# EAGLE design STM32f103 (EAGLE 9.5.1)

## Sheet 1 of 9: STM32F103C8TU
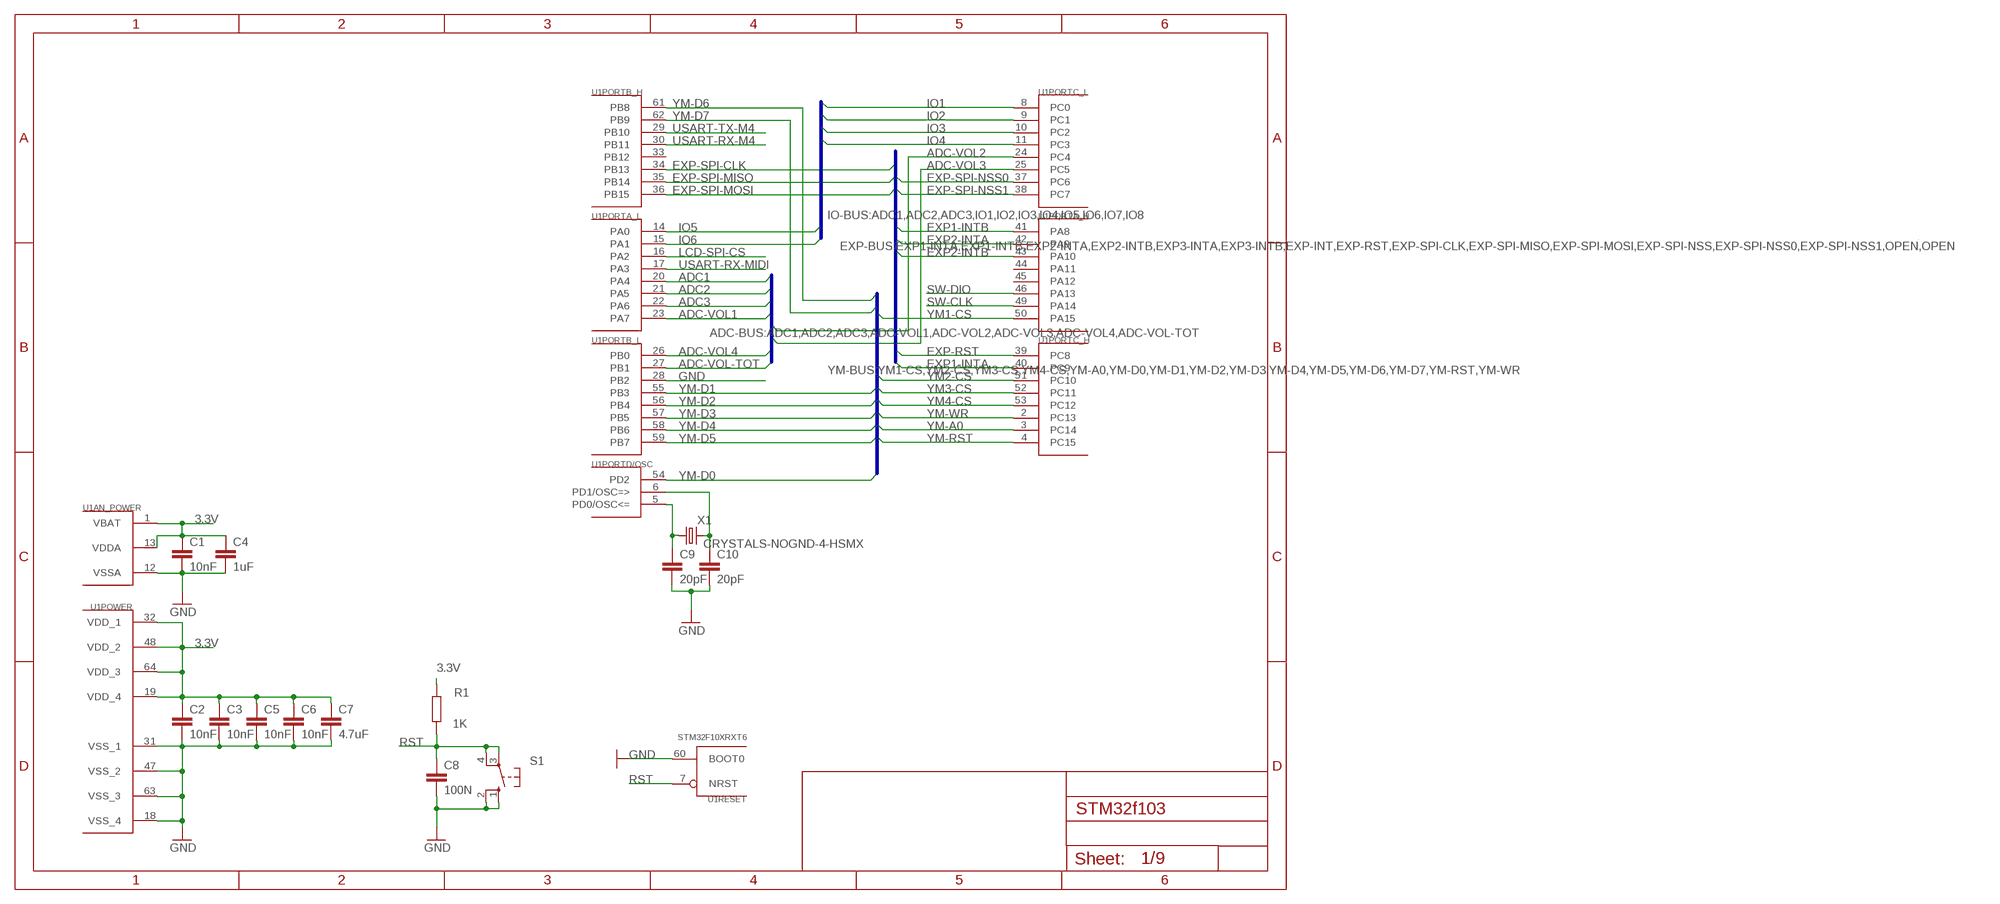
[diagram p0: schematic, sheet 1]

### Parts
C1  10nF  C-EUC0603  [C0603]
C2  10nF  C-EUC0603  [C0603]
C3  10nF  C-EUC0603  [C0603]
C4  1uF  C-EUC0603  [C0603]
C5  10nF  C-EUC0603  [C0603]
C6  10nF  C-EUC0603  [C0603]
C7  4.7uF  C-EUC0603  [C0603]
C8  100N  [0603-SMD]
C9  20pF  C-EUC0603  [C0603]
C10  20pF  C-EUC0603  [C0603]
R1  1K  [0805-SMD]
S1  10-XX  [B3F-10XX]
U1  STM32F10XRXT6  [TQFP64]
X1  CRYSTALS-NOGND-4-HSMX  [HC49-4-HSMX]

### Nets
3.3V: C1.1 C2.1 C3.1 C4.1 C5.1 C6.1 C7.1 R1.2 U1.1(AN_POWER:VBAT) U1.13(AN_POWER:VDDA) U1.19(POWER:VDD_4) U1.32(POWER:VDD_1) U1.48(POWER:VDD_2) U1.64(POWER:VDD_3) ; also sheet 6,9
ADC1: U1.20(PORTA_L:PA4) ; also sheet 9
ADC2: U1.21(PORTA_L:PA5) ; also sheet 9
ADC3: U1.22(PORTA_L:PA6) ; also sheet 9
ADC-VOL1: U1.23(PORTA_L:PA7) ; also sheet 9
ADC-VOL2: U1.24(PORTC_L:PC4) ; also sheet 9
ADC-VOL3: U1.25(PORTC_L:PC5) ; also sheet 9
ADC-VOL4: U1.26(PORTB_L:PB0) ; also sheet 9
ADC-VOL-TOT: U1.27(PORTB_L:PB1) ; also sheet 9
EXP1-INTA: U1.40(PORTC_H:PC9) ; also sheet 9
EXP1-INTB: U1.41(PORTA_H:PA8) ; also sheet 9
EXP2-INTA: U1.42(PORTA_H:PA9) ; also sheet 9
EXP2-INTB: U1.43(PORTA_H:PA10) ; also sheet 9
EXP-RST: U1.39(PORTC_H:PC8) ; also sheet 9
EXP-SPI-CLK: U1.34(PORTB_H:PB13) ; also sheet 9
EXP-SPI-MISO: U1.35(PORTB_H:PB14) ; also sheet 9
EXP-SPI-MOSI: U1.36(PORTB_H:PB15) ; also sheet 9
EXP-SPI-NSS0: U1.37(PORTC_L:PC6) ; also sheet 9
EXP-SPI-NSS1: U1.38(PORTC_L:PC7) ; also sheet 9
GND: C1.2 C2.2 C3.2 C4.2 C5.2 C6.2 C7.2 C8.2 C9.2 C10.2 S1.1(S) S1.2(S1) U1.12(AN_POWER:VSSA) U1.18(POWER:VSS_4) U1.28(PORTB_L:PB2) U1.31(POWER:VSS_1) U1.47(POWER:VSS_2) U1.60(RESET:BOOT0) U1.63(POWER:VSS_3) ; also sheet 2,3,4,5,6,7,8,9
IO1: U1.8(PORTC_L:PC0) ; also sheet 9
IO2: U1.9(PORTC_L:PC1) ; also sheet 9
IO3: U1.10(PORTC_L:PC2) ; also sheet 9
IO4: U1.11(PORTC_L:PC3) ; also sheet 9
IO5: U1.14(PORTA_L:PA0) ; also sheet 9
IO6: U1.15(PORTA_L:PA1) ; also sheet 9
LCD-SPI-CS: U1.16(PORTA_L:PA2) ; also sheet 9
N$1: C9.1 U1.5(PORTD/OSC:PD0/OSC<=) X1.1
N$2: C10.1 U1.6(PORTD/OSC:PD1/OSC=>) X1.2
RST: C8.1 R1.1 S1.3(P) S1.4(P1) U1.7(RESET:NRST)
SW-CLK: U1.49(PORTA_H:PA14) ; also sheet 9
SW-DIO: U1.46(PORTA_H:PA13) ; also sheet 9
USART-RX-M4: U1.30(PORTB_H:PB11) ; also sheet 9
USART-RX-MIDI: U1.17(PORTA_L:PA3) ; also sheet 7
USART-TX-M4: U1.29(PORTB_H:PB10) ; also sheet 9
YM1-CS: U1.50(PORTA_H:PA15) ; also sheet 2
YM2-CS: U1.51(PORTC_H:PC10) ; also sheet 3
YM3-CS: U1.52(PORTC_H:PC11) ; also sheet 4
YM4-CS: U1.53(PORTC_H:PC12) ; also sheet 5
YM-A0: U1.3(PORTC_H:PC14) ; also sheet 2,3,4,5
YM-D0: U1.54(PORTD/OSC:PD2) ; also sheet 2,3,4,5
YM-D1: U1.55(PORTB_L:PB3) ; also sheet 2,3,4,5
YM-D2: U1.56(PORTB_L:PB4) ; also sheet 2,3,4,5
YM-D3: U1.57(PORTB_L:PB5) ; also sheet 2,3,4,5
YM-D4: U1.58(PORTB_L:PB6) ; also sheet 2,3,4,5
YM-D5: U1.59(PORTB_L:PB7) ; also sheet 2,3,4,5
YM-D6: U1.61(PORTB_H:PB8) ; also sheet 2,3,4,5
YM-D7: U1.62(PORTB_H:PB9) ; also sheet 2,3,4,5
YM-RST: U1.4(PORTC_H:PC15) ; also sheet 2,3,4,5
YM-WR: U1.2(PORTC_H:PC13) ; also sheet 2,3,4,5
Unconnected: U1.33(PORTB_H:PB12) U1.44(PORTA_H:PA11) U1.45(PORTA_H:PA12)

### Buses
YM-BUS:YM1-CS,YM2-CS,YM3-CS,YM4-CS,YM-A0,YM-D0,YM-D1,YM-D2,YM-D3,YM-D4,YM-D5,YM-D6,YM-D7,YM-RST,YM-WR
EXP-BUS:EXP1-INTA,EXP1-INTB,EXP2-INTA,EXP2-INTB,EXP3-INTA,EXP3-INTB,EXP-INT,EXP-RST,EXP-SPI-CLK,EXP-SPI-MISO,EXP-SPI-MOSI,EXP-SPI-NSS,EXP-SPI-NSS0,EXP-SPI-NSS1,OPEN!,OPEN
IO-BUS:ADC1,ADC2,ADC3,IO1,IO2,IO3,IO4,IO5,IO6,IO7,IO8
ADC-BUS:ADC1,ADC2,ADC3,ADC-VOL1,ADC-VOL2,ADC-VOL3,ADC-VOL4,ADC-VOL-TOT

## Sheet 2 of 9: YM3812-0
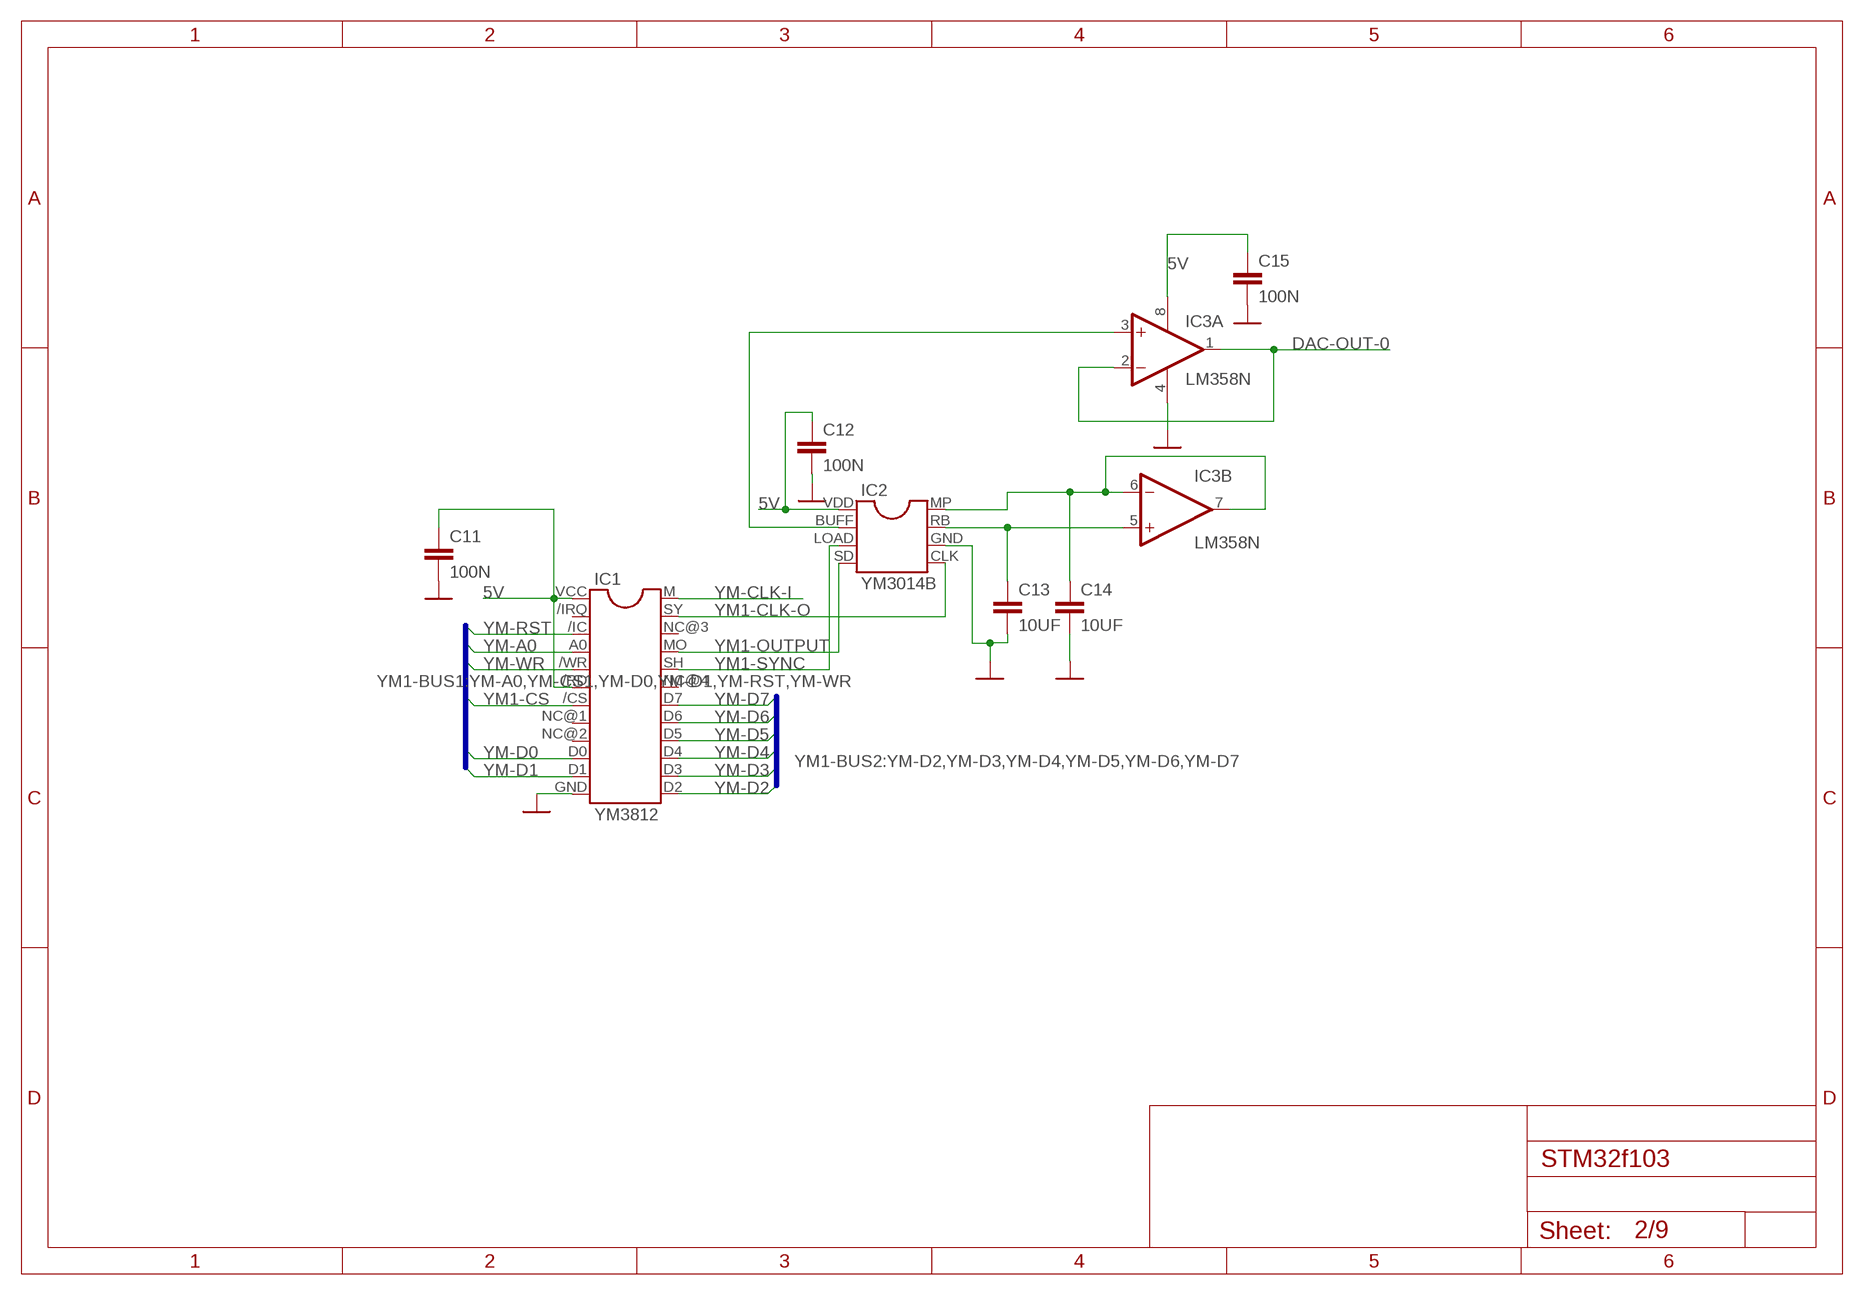
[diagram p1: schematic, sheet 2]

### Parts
C11  100N  [0603-SMD]
C12  100N  [0603-SMD]
C13  10UF  [0603-SMD]
C14  10UF  [0603-SMD]
C15  100N  [0603-SMD]
IC1  YM3812  [YM3812]
IC2  YM3014B  [YM3014B]
IC3  LM358N  [DIL08]

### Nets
5V: C11.1 C12.1 C15.1 IC1./RD IC1.VCC IC2.VDD IC3.8(P:V+) ; also sheet 3,4,5,6,7,8,9
DAC-OUT-0: IC3.1(A:OUT) IC3.2(A:-IN) ; also sheet 9
GND: C11.2 C12.2 C13.2 C14.2 C15.2 IC1.GND IC2.GND IC3.4(P:V-) ; also sheet 1,3,4,5,6,7,8,9
N$3: IC2.BUFF IC3.3(A:+IN)
N$5: C14.1 IC2.MP IC3.6(B:-IN) IC3.7(B:OUT)
N$15: C13.1 IC2.RB IC3.5(B:+IN)
YM1-CLK-O: IC1.SY IC2.CLK ; also sheet 9
YM1-CS: IC1./CS ; also sheet 1
YM1-OUTPUT: IC1.MO IC2.SD ; also sheet 9
YM1-SYNC: IC1.SH IC2.LOAD ; also sheet 9
YM-A0: IC1.A0 ; also sheet 1,3,4,5
YM-CLK-I: IC1.M ; also sheet 3,4,5,8
YM-D0: IC1.D0 ; also sheet 1,3,4,5
YM-D1: IC1.D1 ; also sheet 1,3,4,5
YM-D2: IC1.D2 ; also sheet 1,3,4,5
YM-D3: IC1.D3 ; also sheet 1,3,4,5
YM-D4: IC1.D4 ; also sheet 1,3,4,5
YM-D5: IC1.D5 ; also sheet 1,3,4,5
YM-D6: IC1.D6 ; also sheet 1,3,4,5
YM-D7: IC1.D7 ; also sheet 1,3,4,5
YM-RST: IC1./IC ; also sheet 1,3,4,5
YM-WR: IC1./WR ; also sheet 1,3,4,5
Unconnected: IC1./IRQ IC1.NC@1(NC) IC1.NC@2(NC) IC1.NC@3(NC) IC1.NC@4(NC)

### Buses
YM1-BUS2:YM-D2,YM-D3,YM-D4,YM-D5,YM-D6,YM-D7
YM1-BUS1:YM-A0,YM-CS1,YM-D0,YM-D1,YM-RST,YM-WR

## Sheet 3 of 9: YM3812-1
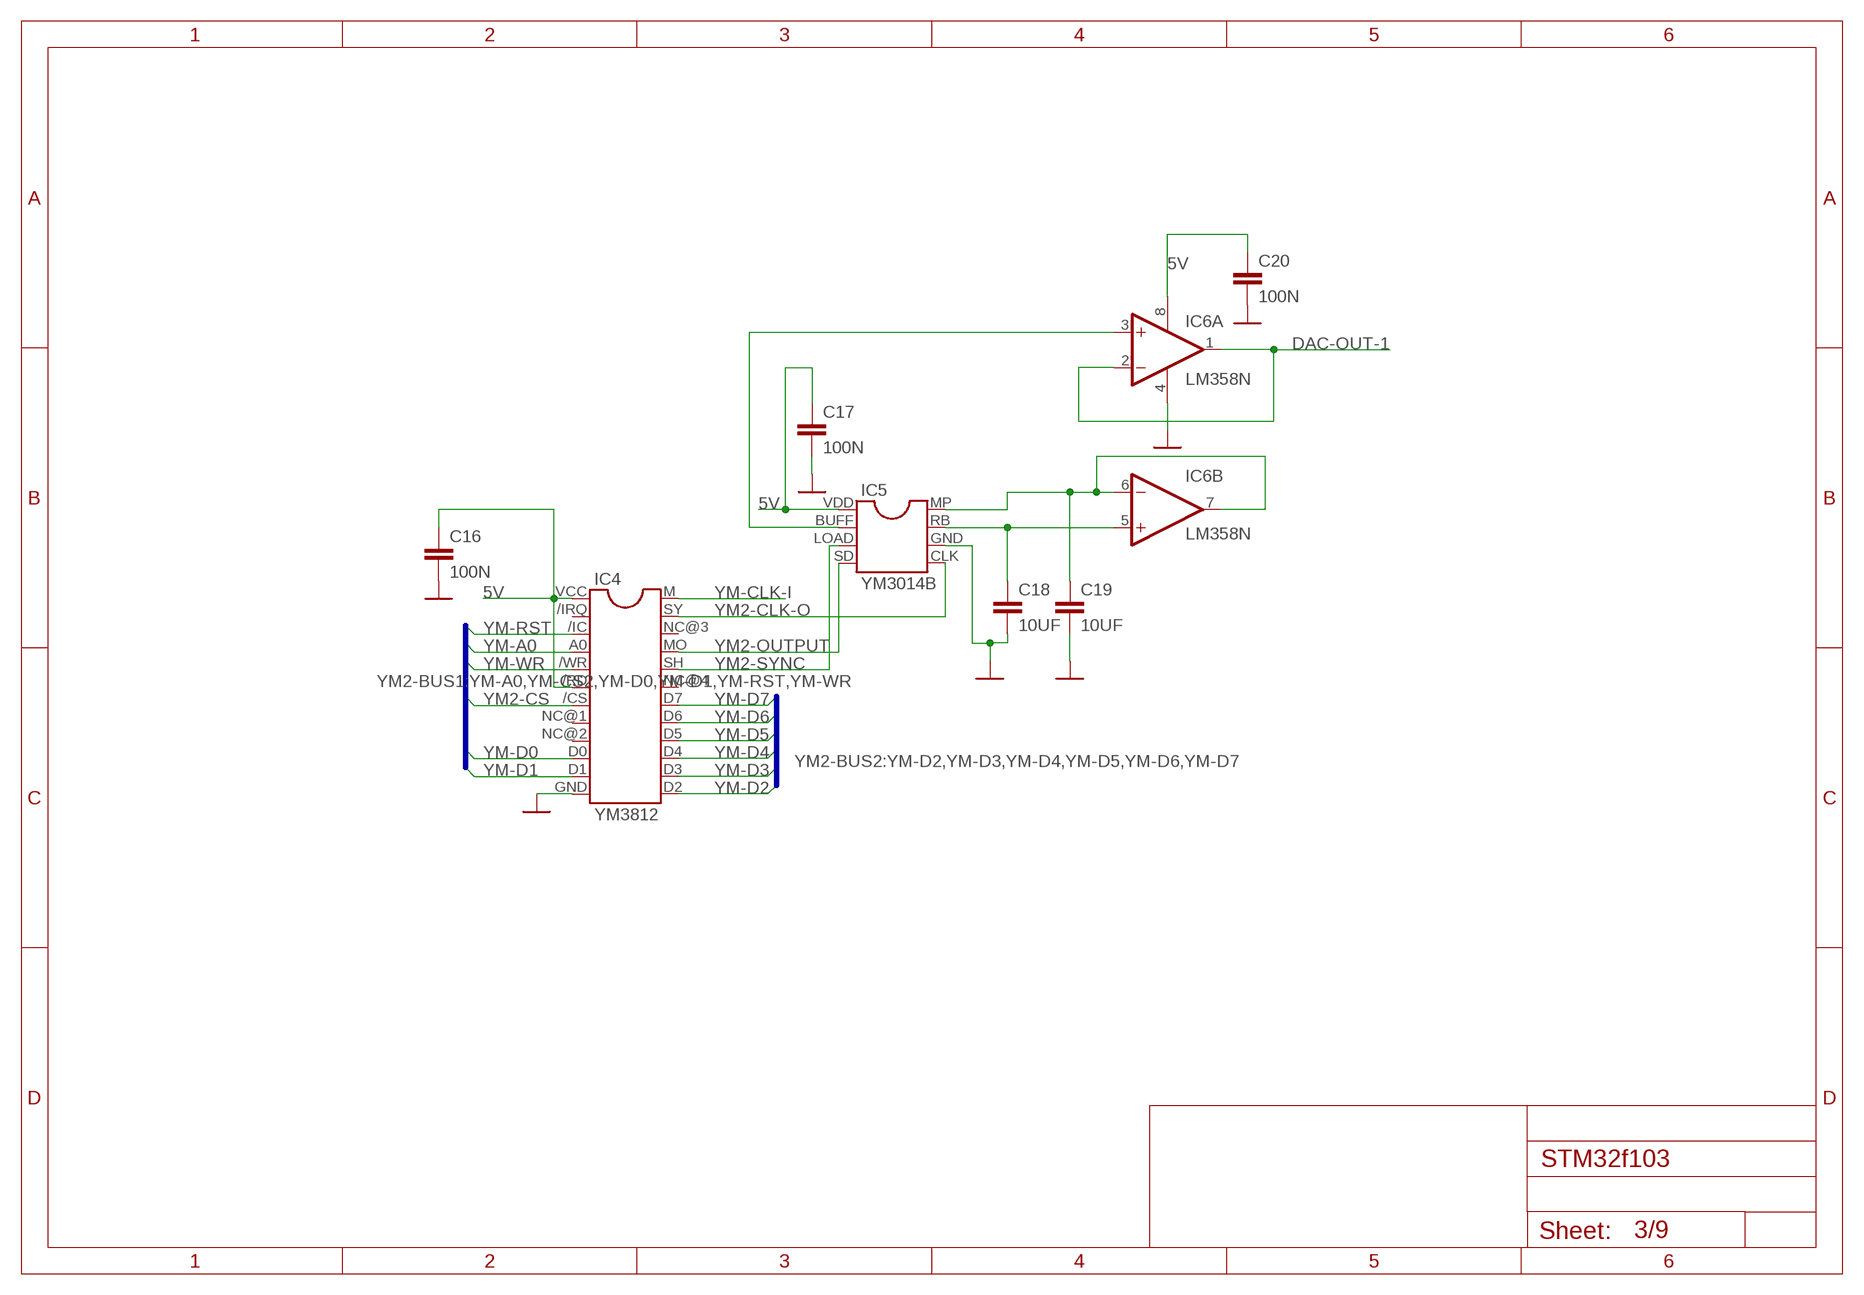
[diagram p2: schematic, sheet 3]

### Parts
C16  100N  [0603-SMD]
C17  100N  [0603-SMD]
C18  10UF  [0603-SMD]
C19  10UF  [0603-SMD]
C20  100N  [0603-SMD]
IC4  YM3812  [YM3812]
IC5  YM3014B  [YM3014B]
IC6  LM358N  [DIL08]

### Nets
5V: C16.1 C17.1 C20.1 IC4./RD IC4.VCC IC5.VDD IC6.8(P:V+) ; also sheet 2,4,5,6,7,8,9
DAC-OUT-1: IC6.1(A:OUT) IC6.2(A:-IN) ; also sheet 9
GND: C16.2 C17.2 C18.2 C19.2 C20.2 IC4.GND IC5.GND IC6.4(P:V-) ; also sheet 1,2,4,5,6,7,8,9
N$4: C18.1 IC5.RB IC6.5(B:+IN)
N$6: IC5.BUFF IC6.3(A:+IN)
N$8: C19.1 IC5.MP IC6.6(B:-IN) IC6.7(B:OUT)
YM2-CLK-O: IC4.SY IC5.CLK ; also sheet 9
YM2-CS: IC4./CS ; also sheet 1
YM2-OUTPUT: IC4.MO IC5.SD ; also sheet 9
YM2-SYNC: IC4.SH IC5.LOAD ; also sheet 9
YM-A0: IC4.A0 ; also sheet 1,2,4,5
YM-CLK-I: IC4.M ; also sheet 2,4,5,8
YM-D0: IC4.D0 ; also sheet 1,2,4,5
YM-D1: IC4.D1 ; also sheet 1,2,4,5
YM-D2: IC4.D2 ; also sheet 1,2,4,5
YM-D3: IC4.D3 ; also sheet 1,2,4,5
YM-D4: IC4.D4 ; also sheet 1,2,4,5
YM-D5: IC4.D5 ; also sheet 1,2,4,5
YM-D6: IC4.D6 ; also sheet 1,2,4,5
YM-D7: IC4.D7 ; also sheet 1,2,4,5
YM-RST: IC4./IC ; also sheet 1,2,4,5
YM-WR: IC4./WR ; also sheet 1,2,4,5
Unconnected: IC4./IRQ IC4.NC@1(NC) IC4.NC@2(NC) IC4.NC@3(NC) IC4.NC@4(NC)

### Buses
YM2-BUS2:YM-D2,YM-D3,YM-D4,YM-D5,YM-D6,YM-D7
YM2-BUS1:YM-A0,YM-CS2,YM-D0,YM-D1,YM-RST,YM-WR

## Sheet 4 of 9: YM3812-2
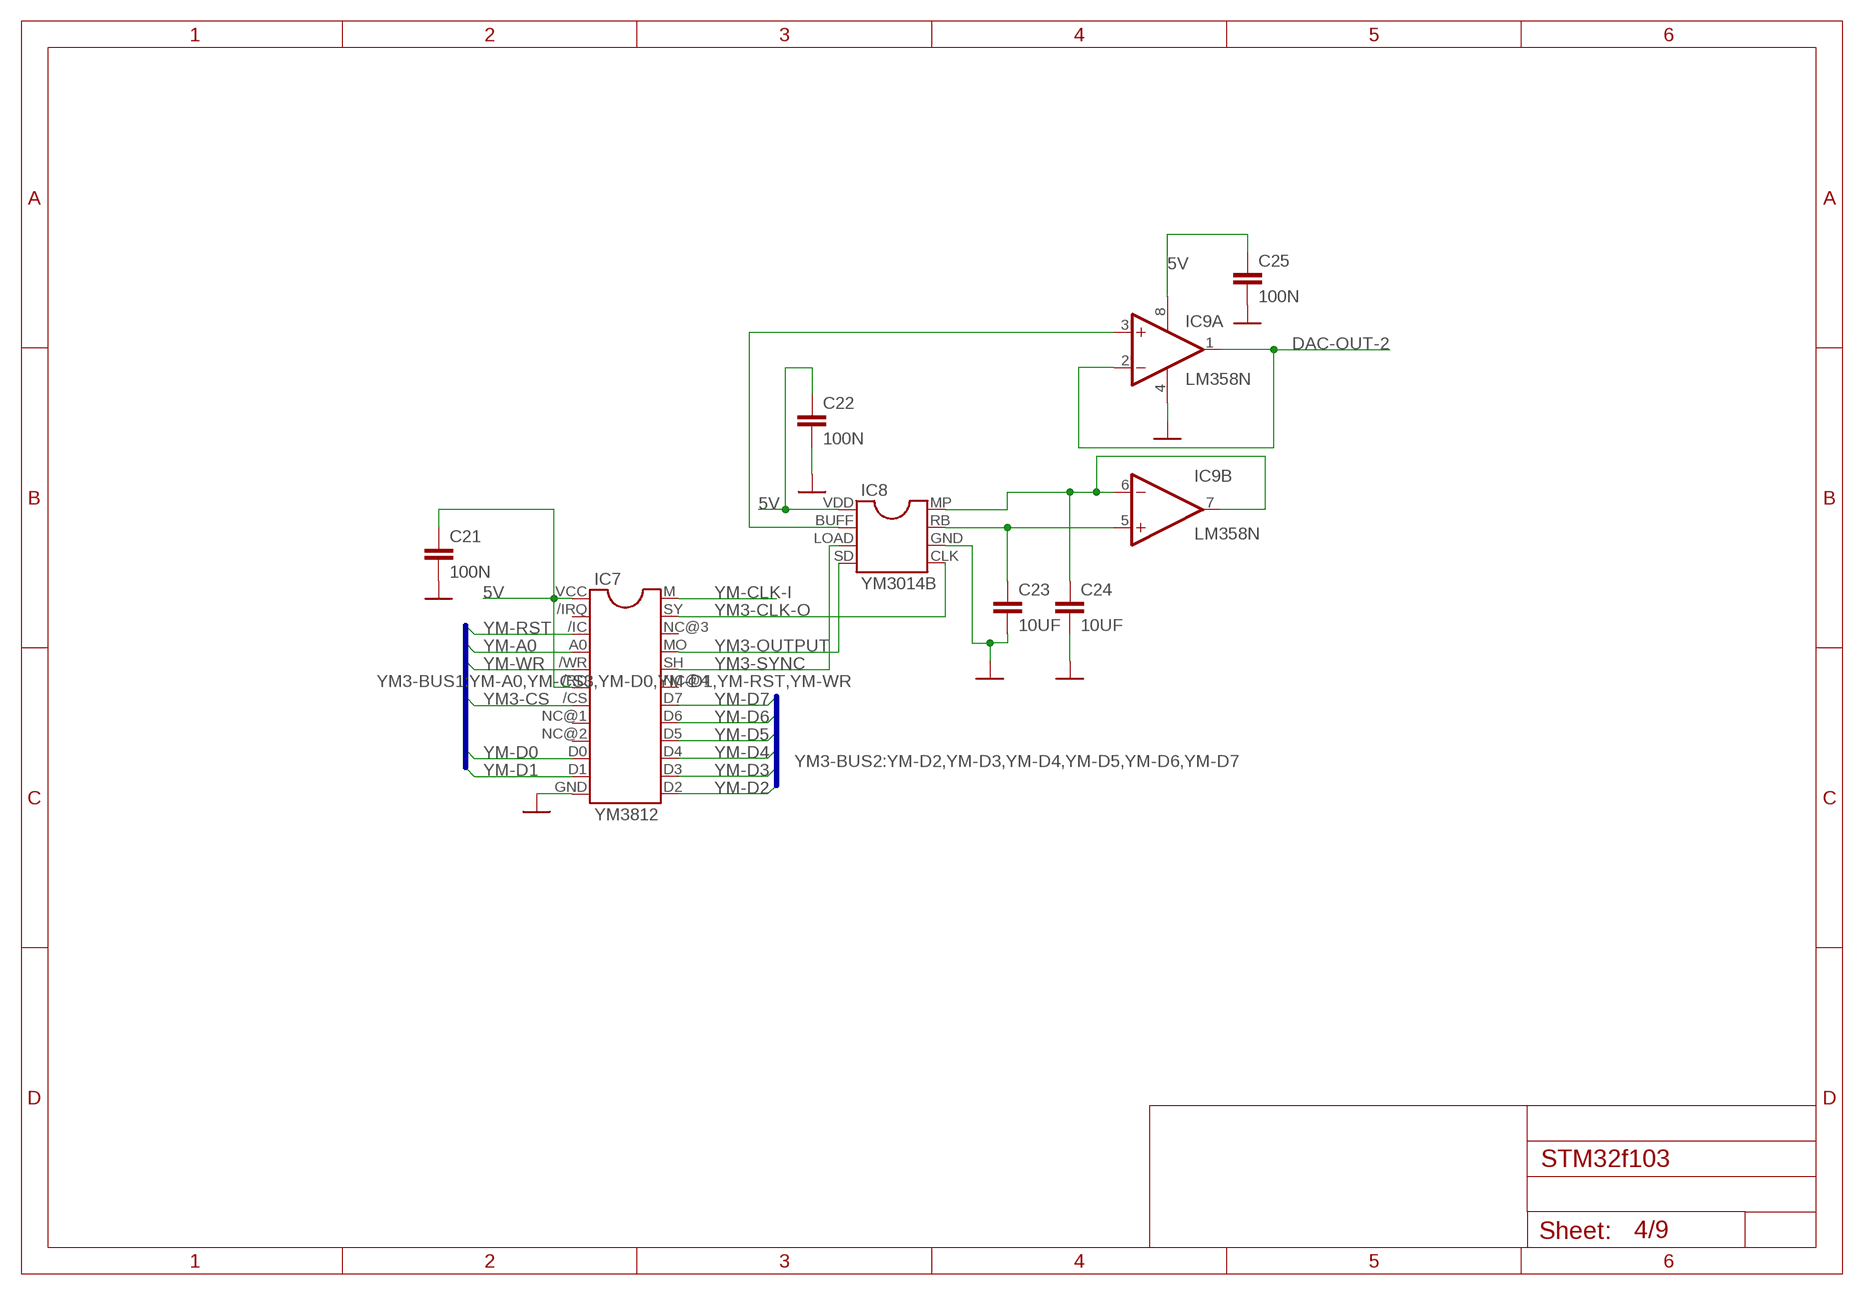
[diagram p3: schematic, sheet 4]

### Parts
C21  100N  [0603-SMD]
C22  100N  [0603-SMD]
C23  10UF  [0603-SMD]
C24  10UF  [0603-SMD]
C25  100N  [0603-SMD]
IC7  YM3812  [YM3812]
IC8  YM3014B  [YM3014B]
IC9  LM358N  [DIL08]

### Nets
5V: C21.1 C22.1 C25.1 IC7./RD IC7.VCC IC8.VDD IC9.8(P:V+) ; also sheet 2,3,5,6,7,8,9
DAC-OUT-2: IC9.1(A:OUT) IC9.2(A:-IN) ; also sheet 9
GND: C21.2 C22.2 C23.2 C24.2 C25.2 IC7.GND IC8.GND IC9.4(P:V-) ; also sheet 1,2,3,5,6,7,8,9
N$7: C23.1 IC8.RB IC9.5(B:+IN)
N$9: IC8.BUFF IC9.3(A:+IN)
N$11: C24.1 IC8.MP IC9.6(B:-IN) IC9.7(B:OUT)
YM3-CLK-O: IC7.SY IC8.CLK ; also sheet 9
YM3-CS: IC7./CS ; also sheet 1
YM3-OUTPUT: IC7.MO IC8.SD ; also sheet 9
YM3-SYNC: IC7.SH IC8.LOAD ; also sheet 9
YM-A0: IC7.A0 ; also sheet 1,2,3,5
YM-CLK-I: IC7.M ; also sheet 2,3,5,8
YM-D0: IC7.D0 ; also sheet 1,2,3,5
YM-D1: IC7.D1 ; also sheet 1,2,3,5
YM-D2: IC7.D2 ; also sheet 1,2,3,5
YM-D3: IC7.D3 ; also sheet 1,2,3,5
YM-D4: IC7.D4 ; also sheet 1,2,3,5
YM-D5: IC7.D5 ; also sheet 1,2,3,5
YM-D6: IC7.D6 ; also sheet 1,2,3,5
YM-D7: IC7.D7 ; also sheet 1,2,3,5
YM-RST: IC7./IC ; also sheet 1,2,3,5
YM-WR: IC7./WR ; also sheet 1,2,3,5
Unconnected: IC7./IRQ IC7.NC@1(NC) IC7.NC@2(NC) IC7.NC@3(NC) IC7.NC@4(NC)

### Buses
YM3-BUS2:YM-D2,YM-D3,YM-D4,YM-D5,YM-D6,YM-D7
YM3-BUS1:YM-A0,YM-CS3,YM-D0,YM-D1,YM-RST,YM-WR

## Sheet 5 of 9: YM3812-3
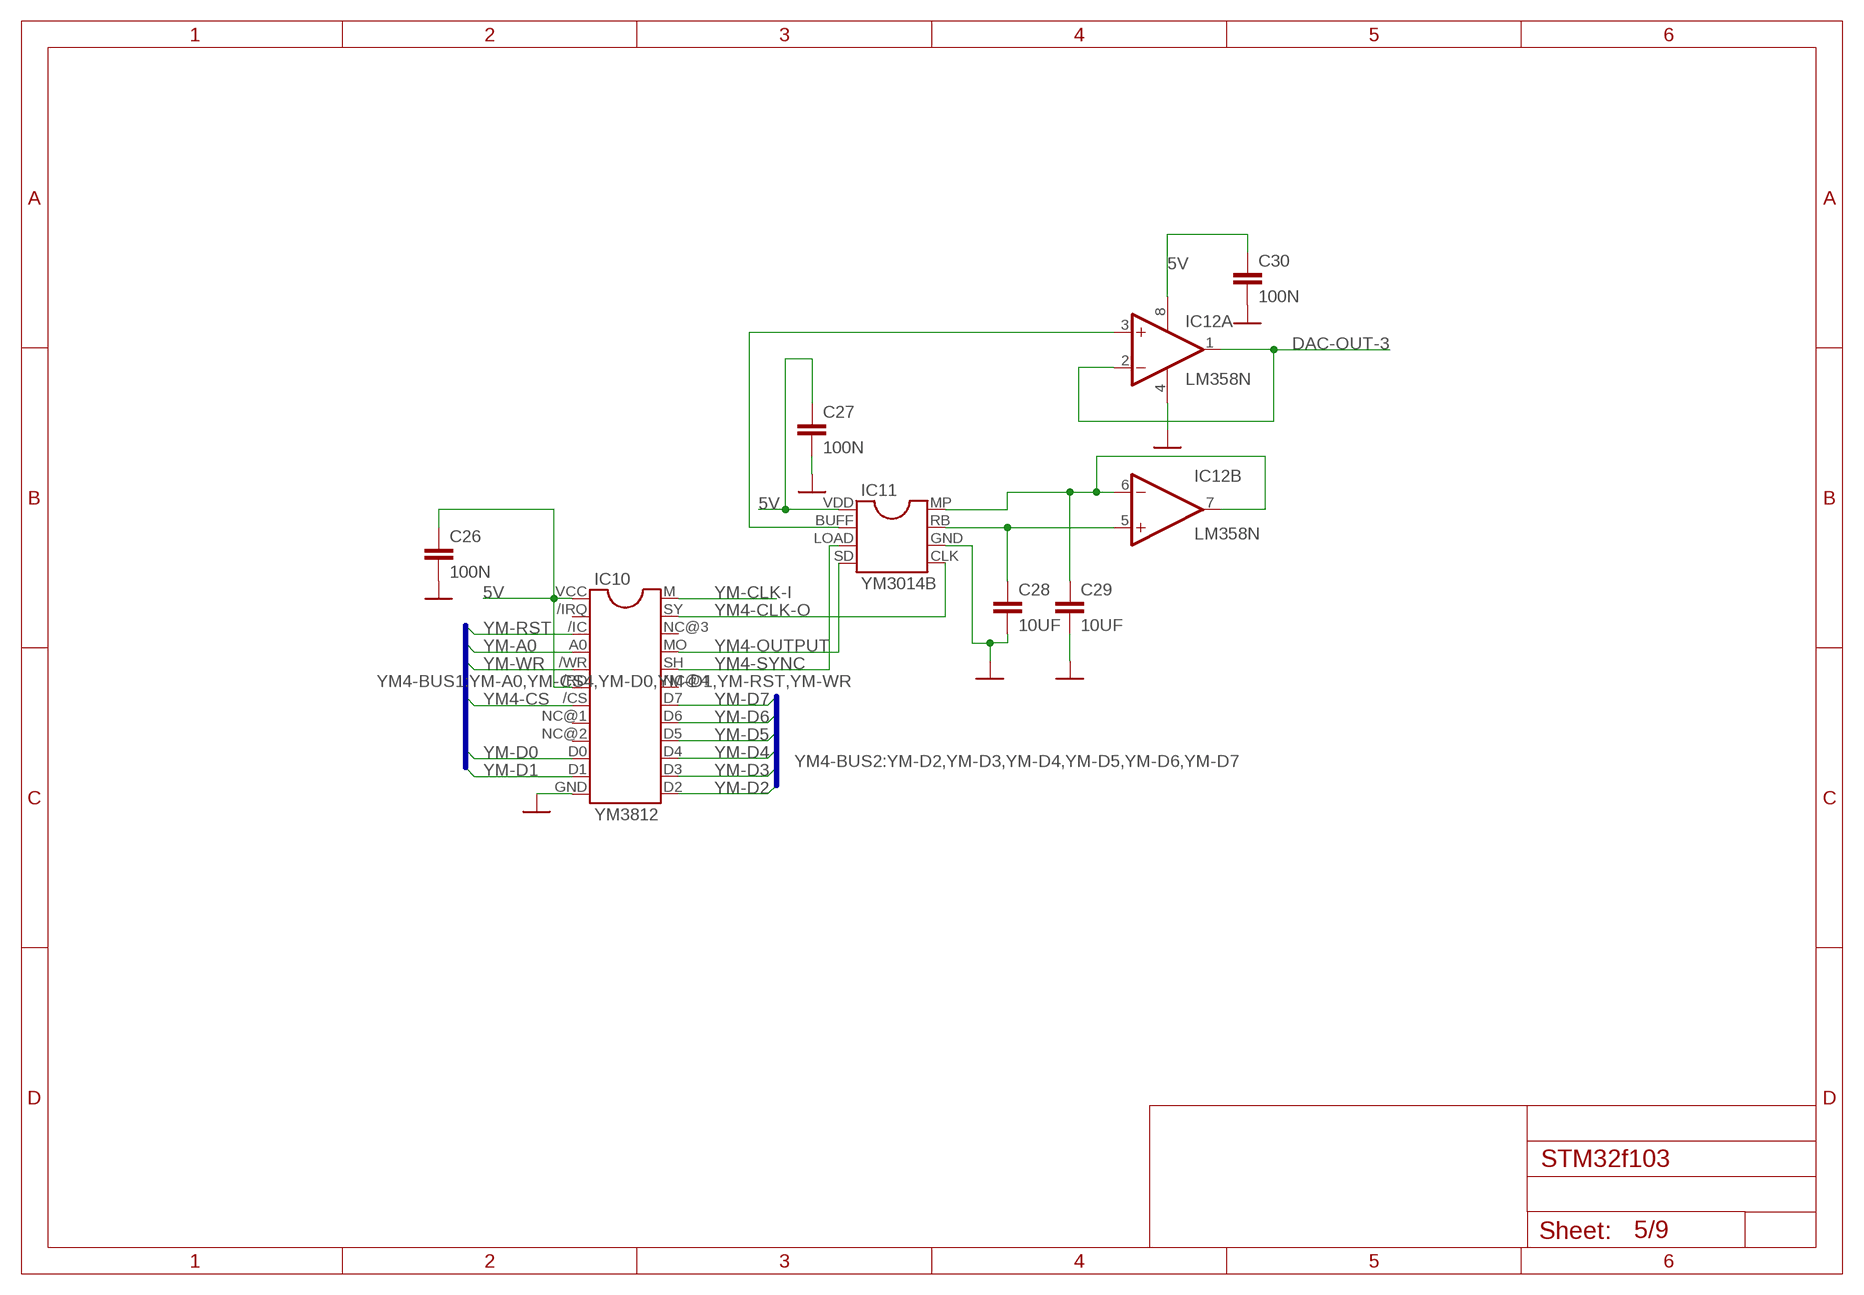
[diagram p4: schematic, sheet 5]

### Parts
C26  100N  [0603-SMD]
C27  100N  [0603-SMD]
C28  10UF  [0603-SMD]
C29  10UF  [0603-SMD]
C30  100N  [0603-SMD]
IC10  YM3812  [YM3812]
IC11  YM3014B  [YM3014B]
IC12  LM358N  [DIL08]

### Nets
5V: C26.1 C27.1 C30.1 IC10./RD IC10.VCC IC11.VDD IC12.8(P:V+) ; also sheet 2,3,4,6,7,8,9
DAC-OUT-3: IC12.1(A:OUT) IC12.2(A:-IN) ; also sheet 9
GND: C26.2 C27.2 C28.2 C29.2 C30.2 IC10.GND IC11.GND IC12.4(P:V-) ; also sheet 1,2,3,4,6,7,8,9
N$10: C28.1 IC11.RB IC12.5(B:+IN)
N$12: IC11.BUFF IC12.3(A:+IN)
N$14: C29.1 IC11.MP IC12.6(B:-IN) IC12.7(B:OUT)
YM4-CLK-O: IC10.SY IC11.CLK ; also sheet 9
YM4-CS: IC10./CS ; also sheet 1
YM4-OUTPUT: IC10.MO IC11.SD ; also sheet 9
YM4-SYNC: IC10.SH IC11.LOAD ; also sheet 9
YM-A0: IC10.A0 ; also sheet 1,2,3,4
YM-CLK-I: IC10.M ; also sheet 2,3,4,8
YM-D0: IC10.D0 ; also sheet 1,2,3,4
YM-D1: IC10.D1 ; also sheet 1,2,3,4
YM-D2: IC10.D2 ; also sheet 1,2,3,4
YM-D3: IC10.D3 ; also sheet 1,2,3,4
YM-D4: IC10.D4 ; also sheet 1,2,3,4
YM-D5: IC10.D5 ; also sheet 1,2,3,4
YM-D6: IC10.D6 ; also sheet 1,2,3,4
YM-D7: IC10.D7 ; also sheet 1,2,3,4
YM-RST: IC10./IC ; also sheet 1,2,3,4
YM-WR: IC10./WR ; also sheet 1,2,3,4
Unconnected: IC10./IRQ IC10.NC@1(NC) IC10.NC@2(NC) IC10.NC@3(NC) IC10.NC@4(NC)

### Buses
YM4-BUS2:YM-D2,YM-D3,YM-D4,YM-D5,YM-D6,YM-D7
YM4-BUS1:YM-A0,YM-CS4,YM-D0,YM-D1,YM-RST,YM-WR

## Sheet 6 of 9: POWER SUPPLY
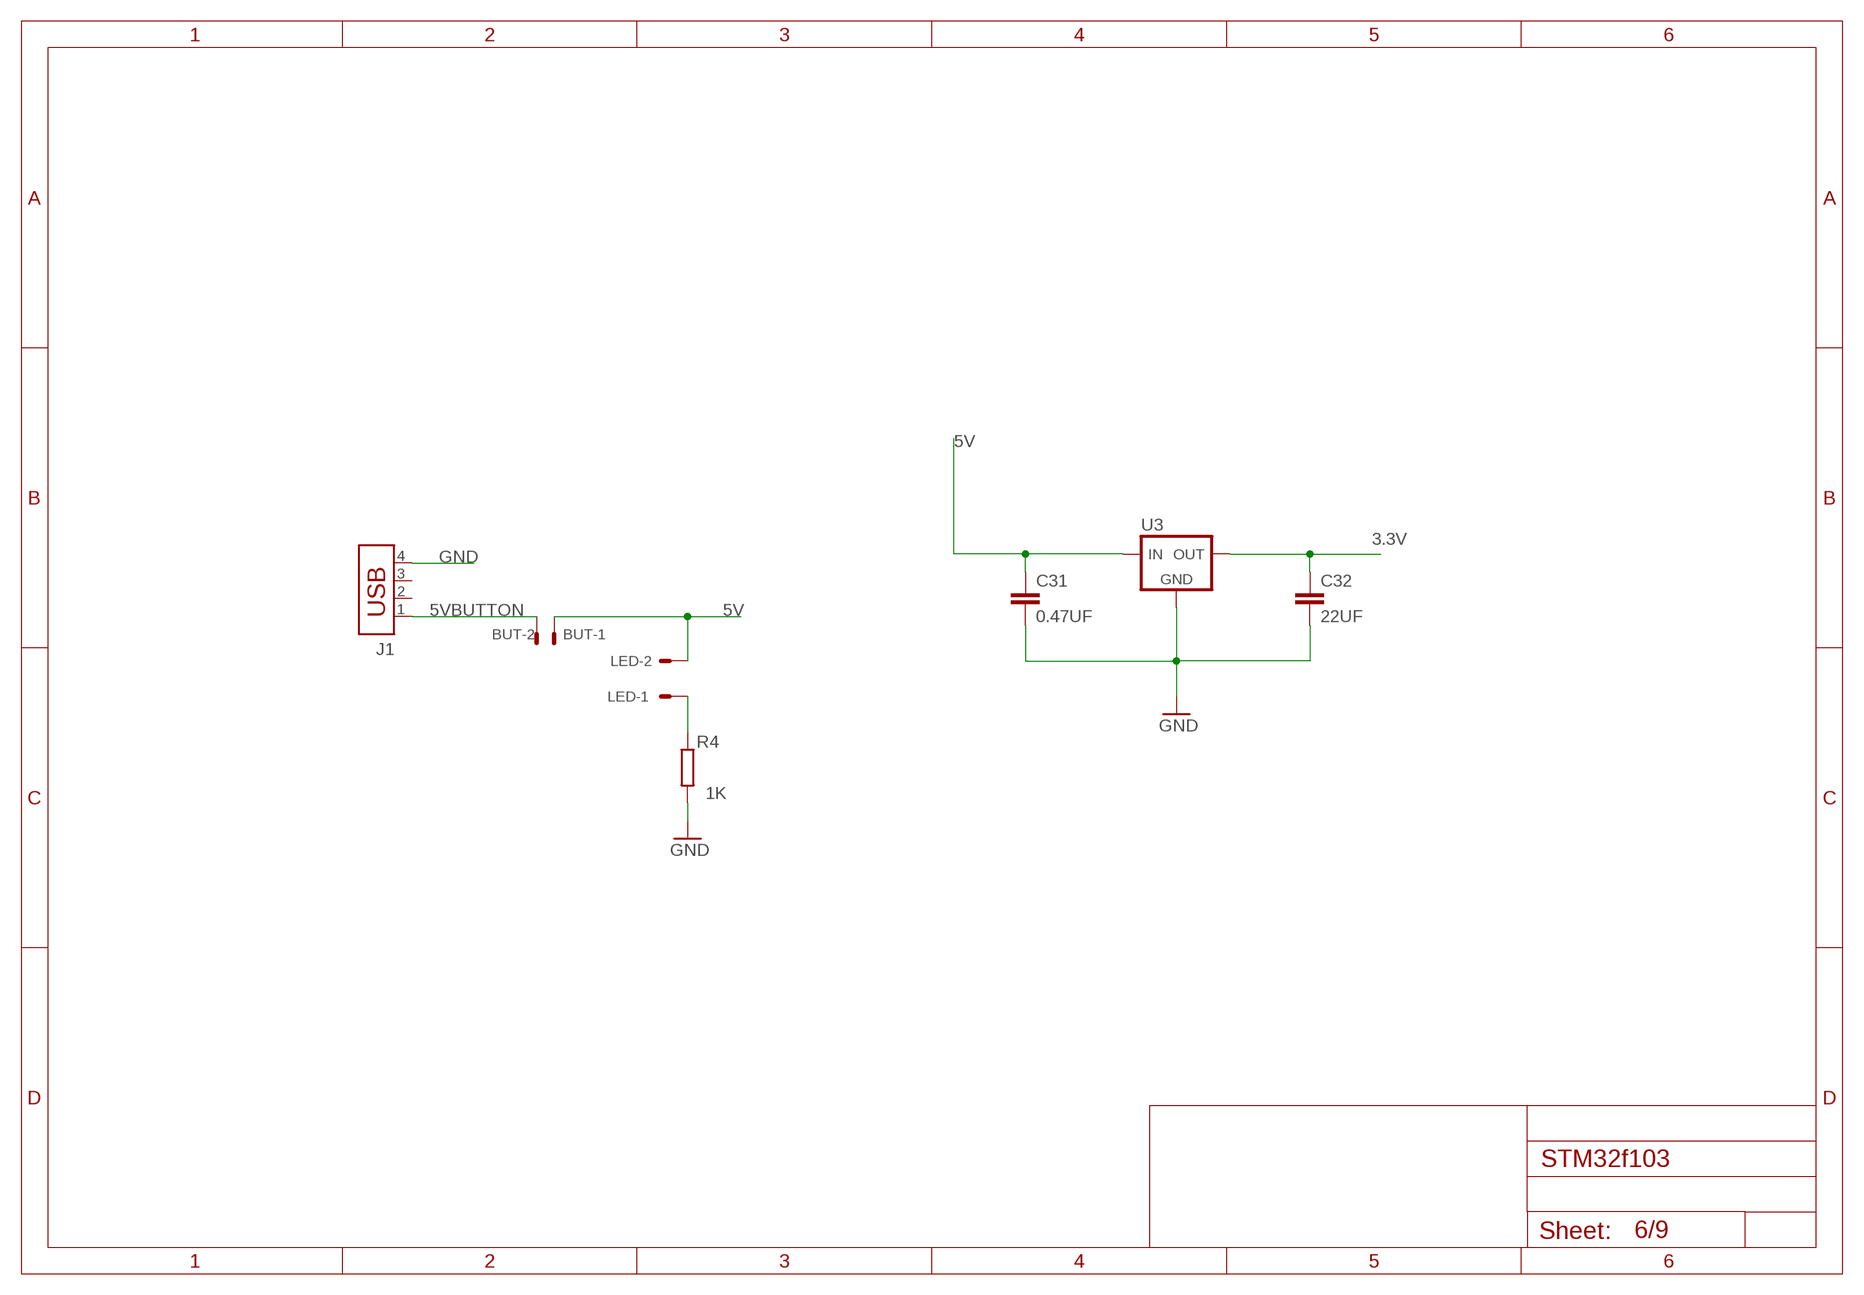
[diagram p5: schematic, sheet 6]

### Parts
BUT  22-27-2021-02  [6410-02]
C31  0.47UF  [0603-SMD]
C32  22UF  [0603-SMD]
J1  CON-USB-B  [USB-B]
LED  22-27-2021-02  [6410-02]
R4  1K  [0805-SMD]
U3  LM2931AT-H  [TO220BH]

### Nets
3.3V: C32.1 U3.3(VOUT) ; also sheet 1,9
5V: BUT.1 C31.1 LED.2 U3.1(VIN) ; also sheet 2,3,4,5,7,8,9
5VBUTTON: BUT.2 J1.1
GND: C31.2 C32.2 J1.4 R4.2 U3.2(GND) ; also sheet 1,2,3,4,5,7,8,9
N$13: LED.1 R4.1
Unconnected: J1.2 J1.3

## Sheet 7 of 9: MIDI
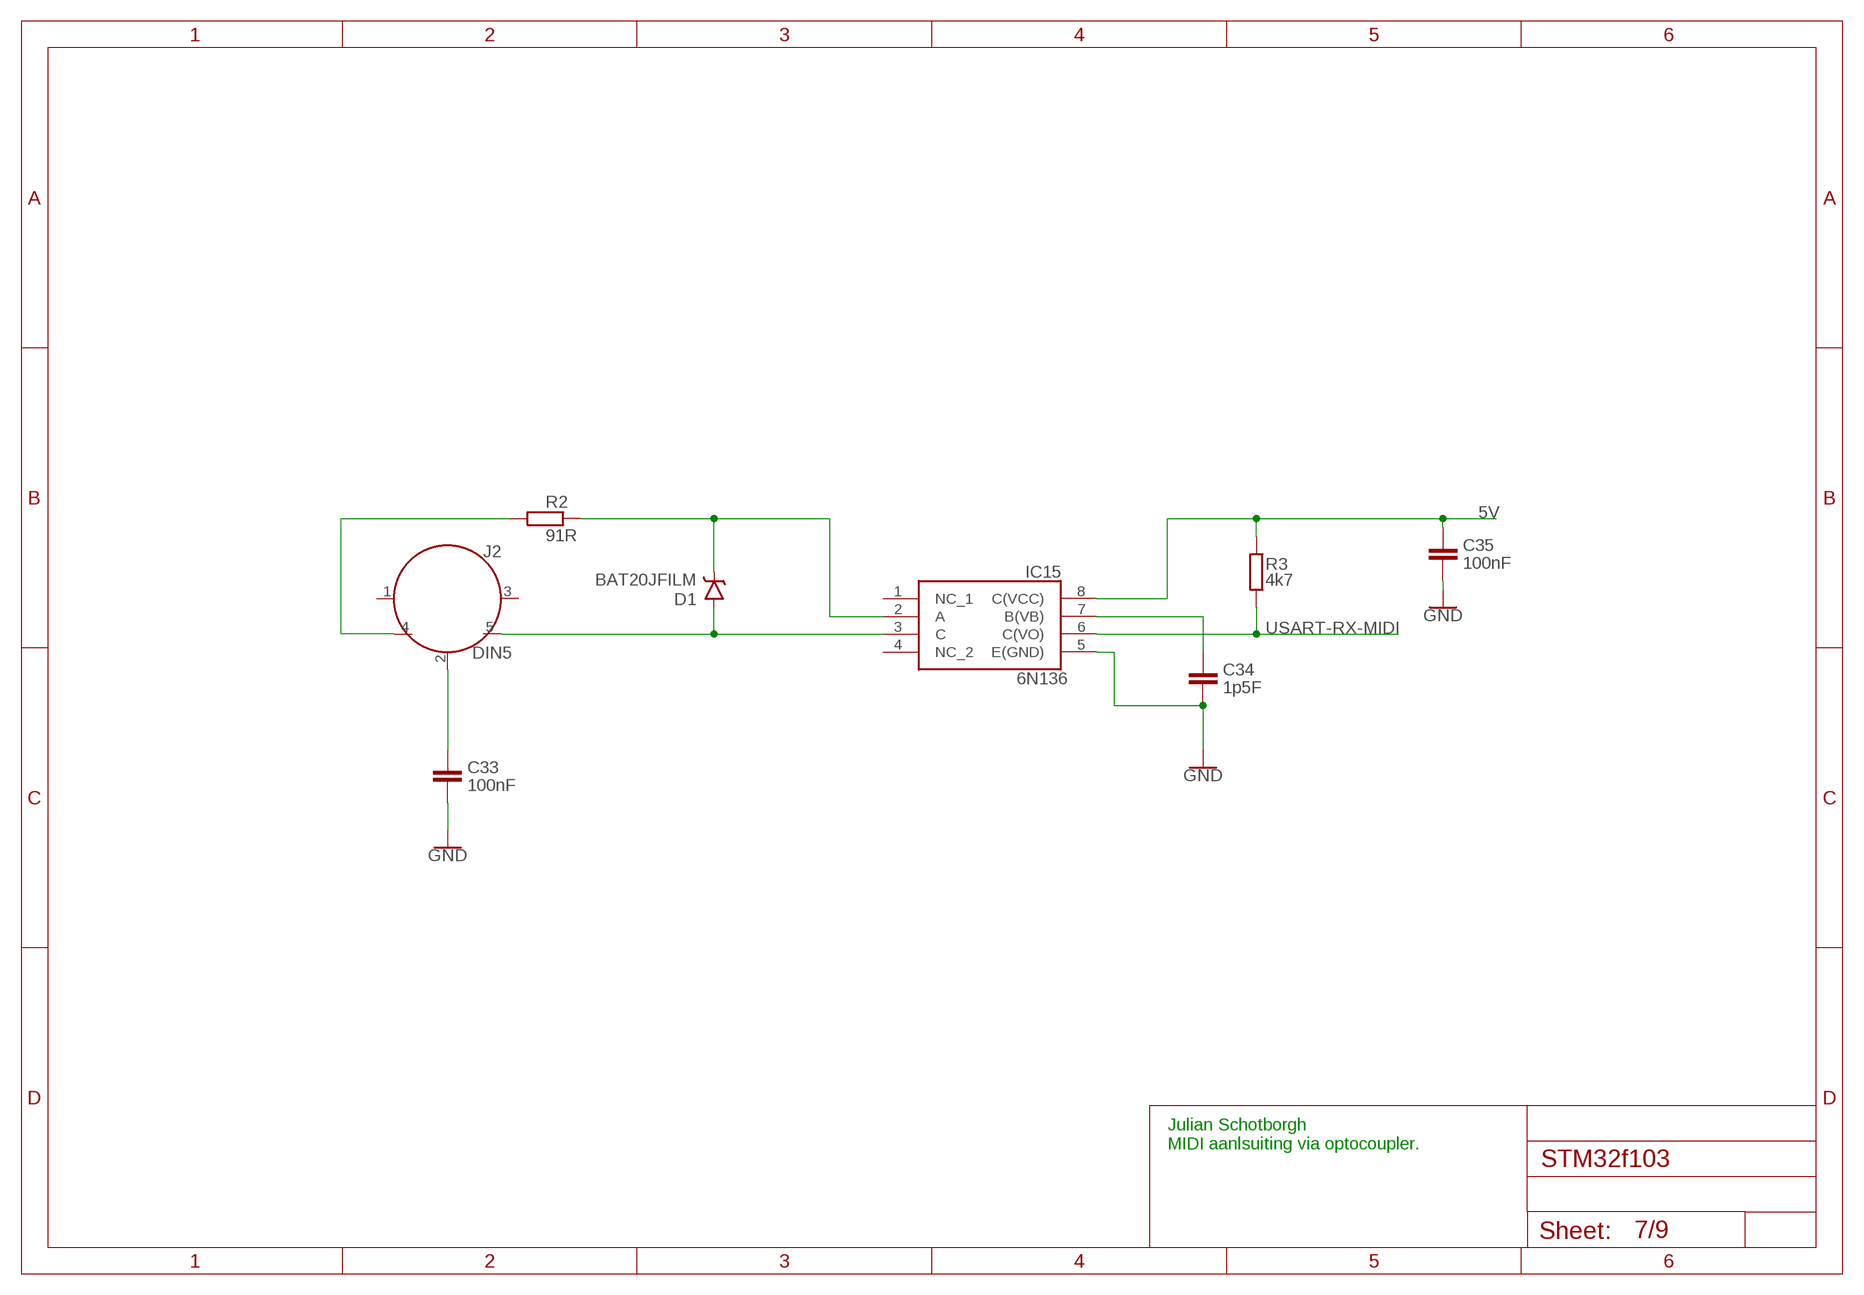
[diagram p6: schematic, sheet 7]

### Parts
C33  100nF  C-EUC0603  [C0603]
C34  1p5F  C-EUC0603  [C0603]
C35  100nF  C-EUC0603  [C0603]
D1  BAT20JFILM  [SOD-323]
IC15  6N136  [DIP762W60P254L1060H465Q8N]
J2  DIN5  [DIN5-RA-PTH]
R2  91R  1K  [0805-SMD]
R3  4k7  1K  [0805-SMD]

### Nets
5V: C35.2 IC15.8(C(VCC)) R3.1 ; also sheet 2,3,4,5,6,8,9
GND: C33.2 C34.1 C35.1 IC15.5(E(GND)) ; also sheet 1,2,3,4,5,6,8,9
N$16: D1.A IC15.3(C) J2.5
N$17: D1.C IC15.2(A) R2.2
N$18: C33.1 J2.2
N$19: J2.4 R2.1
N$21: C34.2 IC15.7(B(VB))
USART-RX-MIDI: IC15.6(C(VO)) R3.2 ; also sheet 1
Unconnected: IC15.1(NC_1) IC15.4(NC_2) J2.1 J2.3

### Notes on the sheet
- Julian Schotborgh
  MIDI aanlsuiting via optocoupler.

## Sheet 8 of 9: YM3812 KLOK
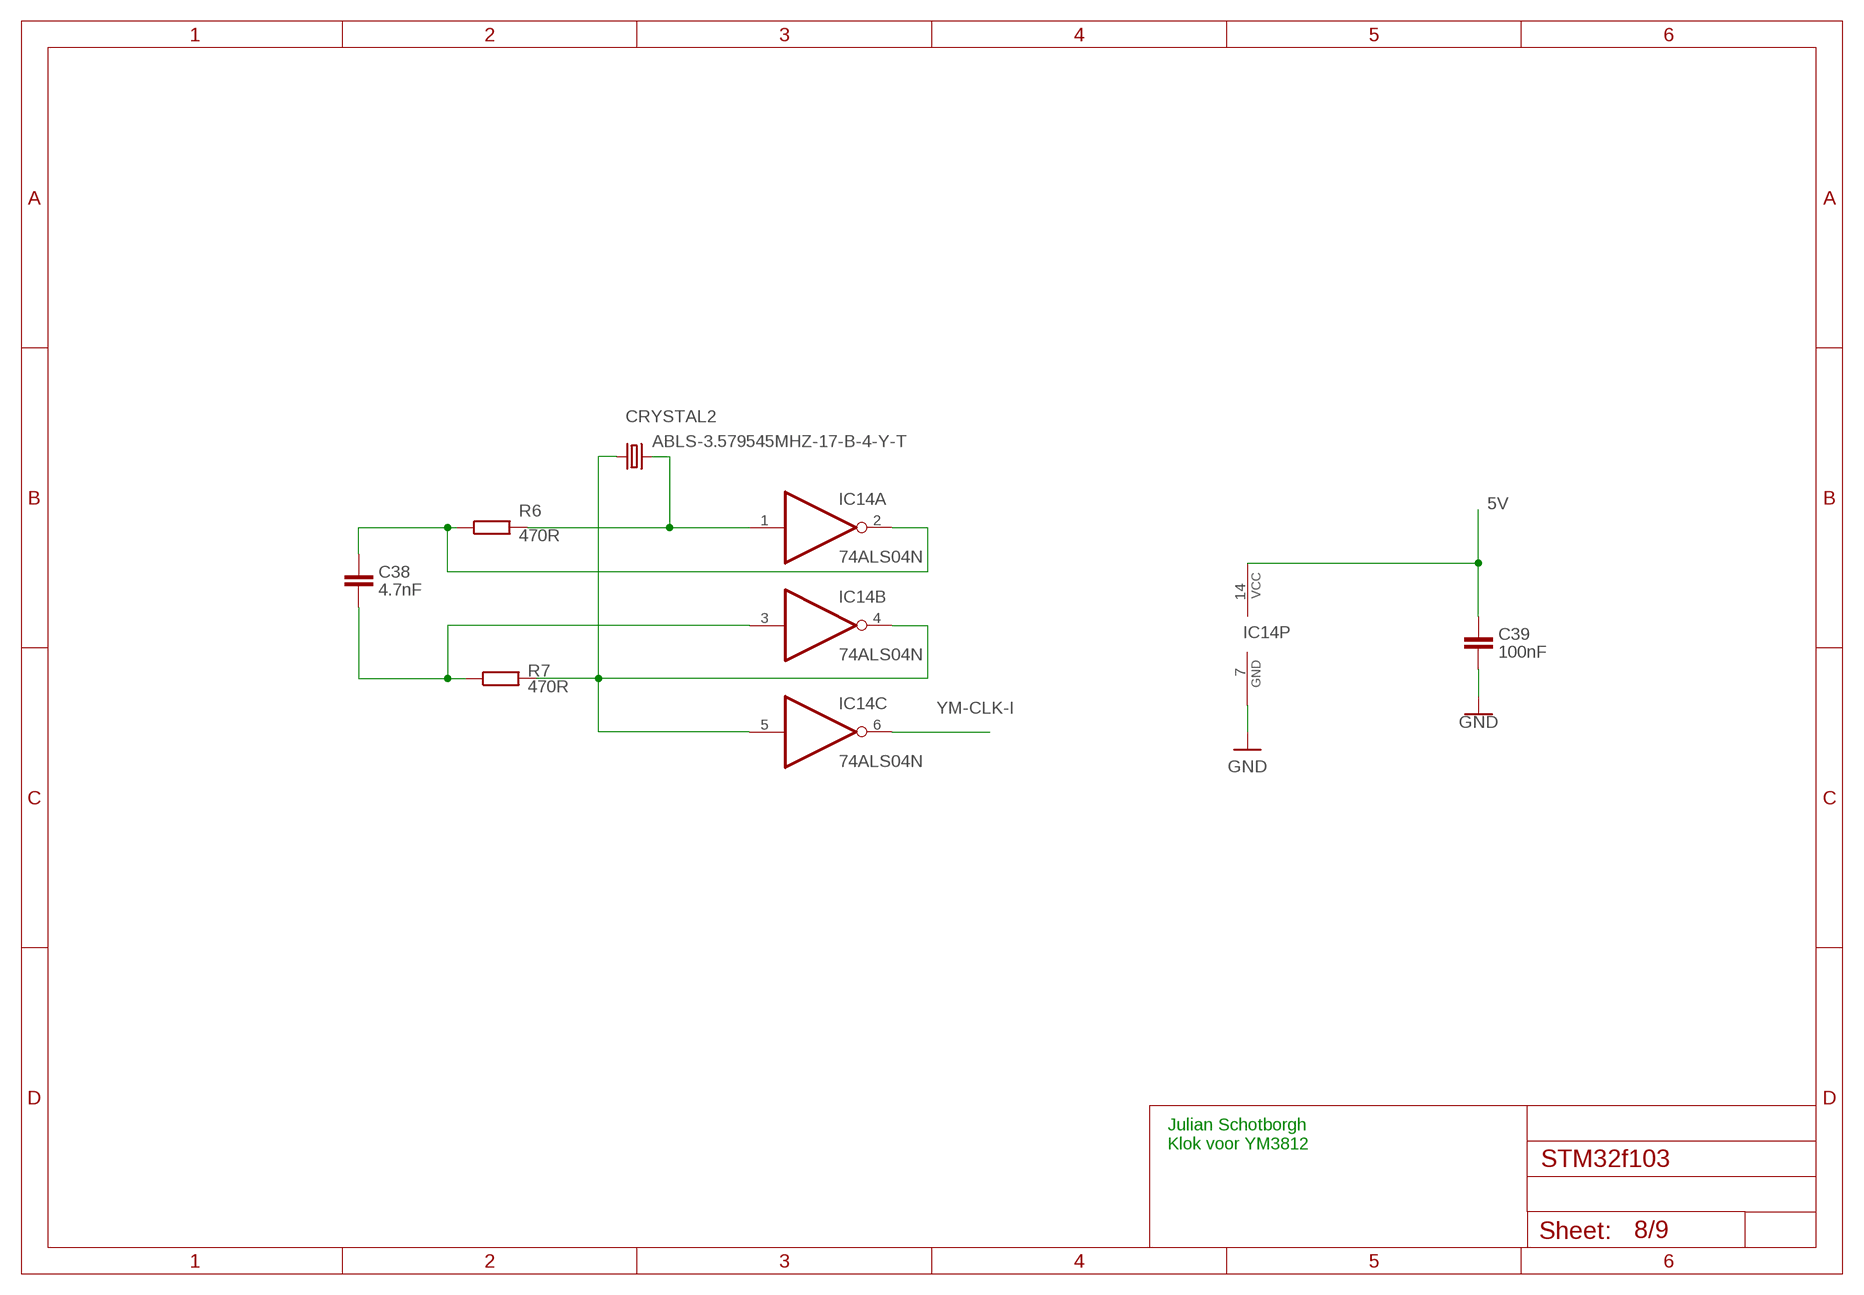
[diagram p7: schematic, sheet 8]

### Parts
C38  4.7nF  C-EUC0603  [C0603]
C39  100nF  C-EUC0603  [C0603]
CRYSTAL2  ABLS-3.579545MHZ-17-B-4-Y-T  [ABLS-3.579545MHZ-17-B-4-Y-T-11.5X4.7X4.2]
IC14  74ALS04N  [DIL14]
R6  470R  1K  [0805-SMD]
R7  470R  1K  [0805-SMD]

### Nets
5V: C39.2 IC14.14(P:VCC) ; also sheet 2,3,4,5,6,7,9
GND: C39.1 IC14.7(P:GND) ; also sheet 1,2,3,4,5,6,7,9
N$20: CRYSTAL2.P$1 IC14.4(B:O) IC14.5(C:I) R7.2
N$25: C38.2 IC14.2(A:O) R6.1
N$26: C38.1 IC14.3(B:I) R7.1
N$27: CRYSTAL2.P$2 IC14.1(A:I) R6.2
YM-CLK-I: IC14.6(C:O) ; also sheet 2,3,4,5
Unconnected: IC14.8(D:O) IC14.9(D:I) IC14.10(E:O) IC14.11(E:I) IC14.12(F:O) IC14.13(F:I)

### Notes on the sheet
- Julian Schotborgh
  Klok voor YM3812

## Sheet 9 of 9: OUTPUTS-EXP/ADC/HEADERS
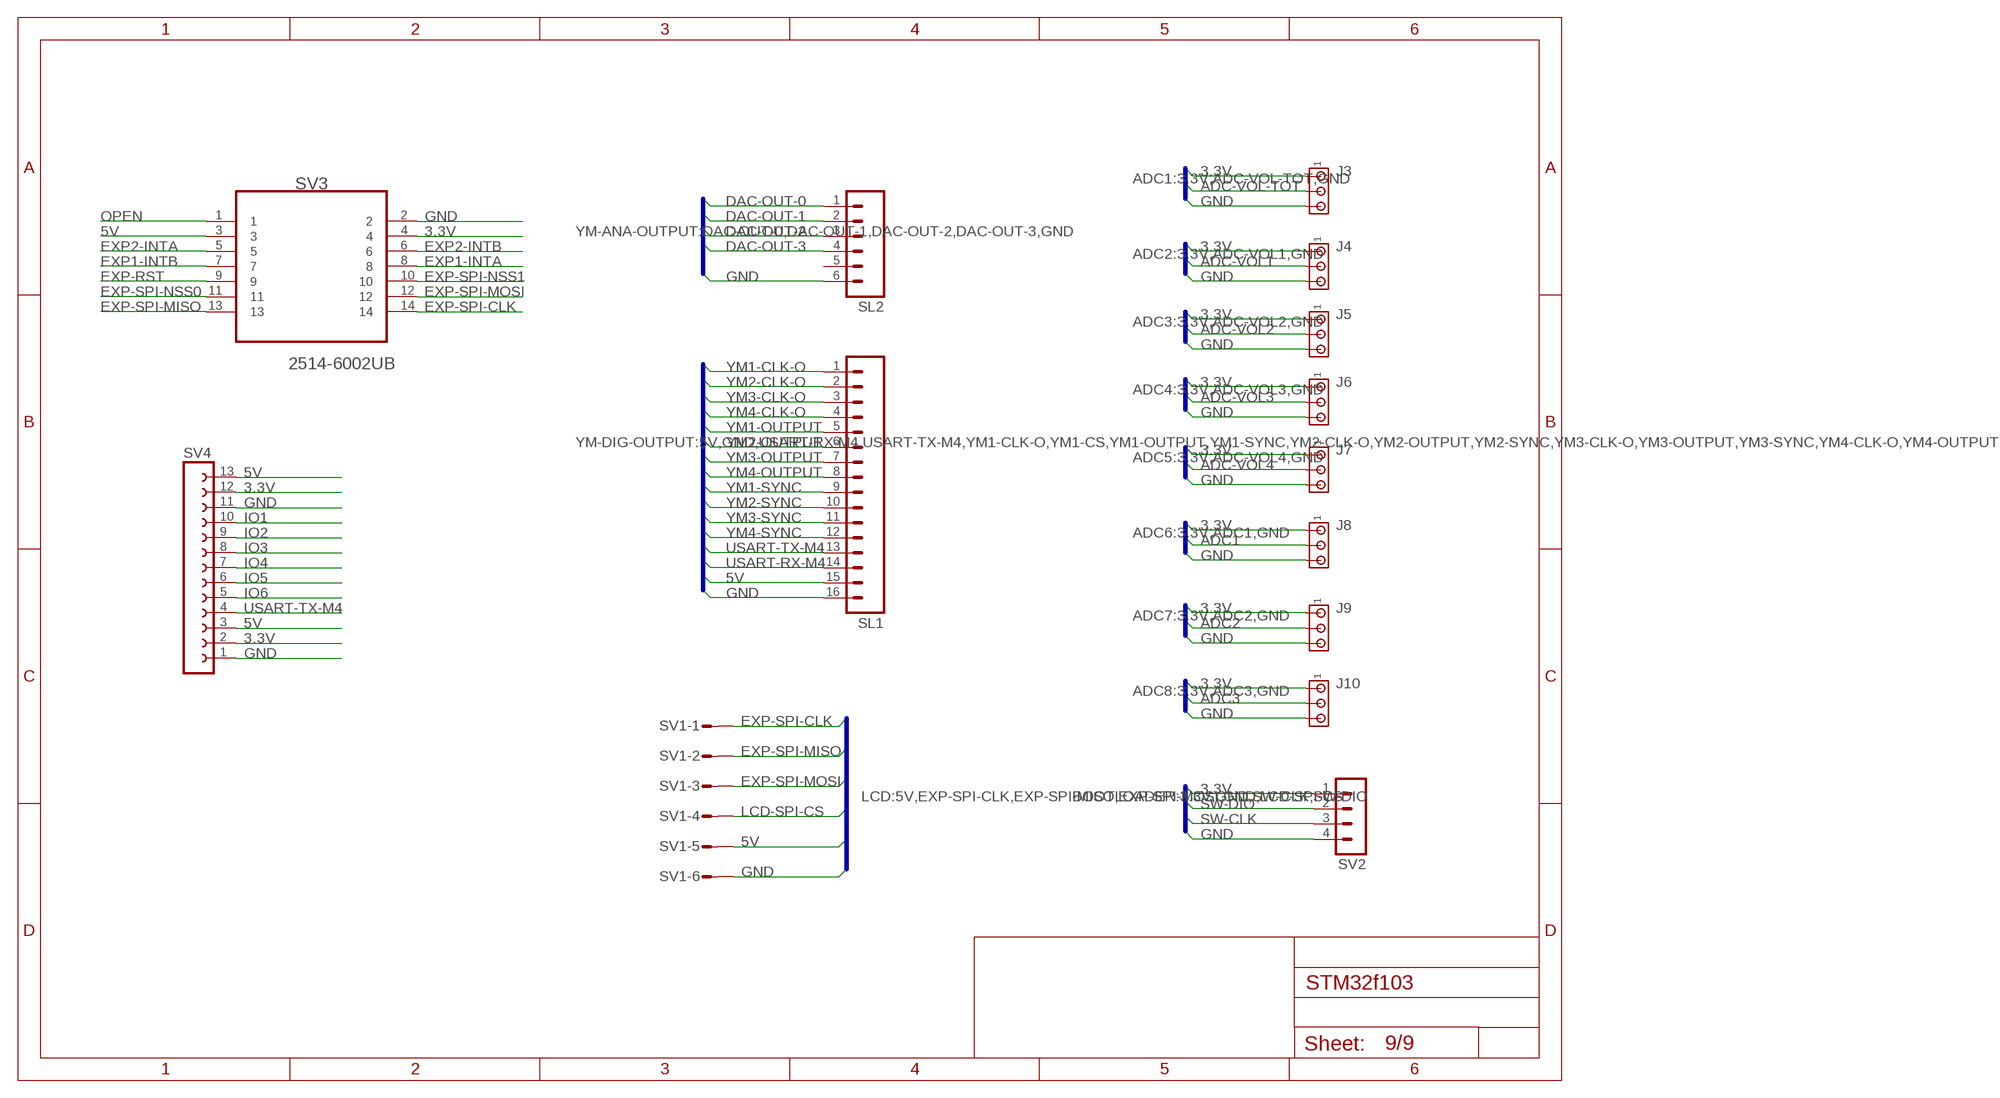
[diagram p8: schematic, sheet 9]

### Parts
J3  MTA03-156  [1X3MTA]
J4  MTA03-156  [1X3MTA]
J5  MTA03-156  [1X3MTA]
J6  MTA03-156  [1X3MTA]
J7  MTA03-156  [1X3MTA]
J8  MTA03-156  [1X3MTA]
J9  MTA03-156  [1X3MTA]
J10  MTA03-156  [1X3MTA]
SL1  M16  [16P]
SL2  M06  [06P]
SV1  S06P  [S06P]
SV2  MA04-1  [MA04-1]
SV3  2514-6002UB  [3M_2514-6002UB]
SV4  FE13-1  [FE13]

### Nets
3.3V: J3.1 J4.1 J5.1 J6.1 J7.1 J8.1 J9.1 J10.1 SV2.1 SV3.4 SV4.2 SV4.12 ; also sheet 1,6
5V: SL1.15 SV1.5 SV3.3 SV4.3 SV4.13 ; also sheet 2,3,4,5,6,7,8
ADC1: J8.2 ; also sheet 1
ADC2: J9.2 ; also sheet 1
ADC3: J10.2 ; also sheet 1
ADC-VOL1: J4.2 ; also sheet 1
ADC-VOL2: J5.2 ; also sheet 1
ADC-VOL3: J6.2 ; also sheet 1
ADC-VOL4: J7.2 ; also sheet 1
ADC-VOL-TOT: J3.2 ; also sheet 1
DAC-OUT-0: SL2.1 ; also sheet 2
DAC-OUT-1: SL2.2 ; also sheet 3
DAC-OUT-2: SL2.3 ; also sheet 4
DAC-OUT-3: SL2.4 ; also sheet 5
EXP1-INTA: SV3.8 ; also sheet 1
EXP1-INTB: SV3.7 ; also sheet 1
EXP2-INTA: SV3.5 ; also sheet 1
EXP2-INTB: SV3.6 ; also sheet 1
EXP-RST: SV3.9 ; also sheet 1
EXP-SPI-CLK: SV1.1 SV3.14 ; also sheet 1
EXP-SPI-MISO: SV1.2 SV3.13 ; also sheet 1
EXP-SPI-MOSI: SV1.3 SV3.12 ; also sheet 1
EXP-SPI-NSS0: SV3.11 ; also sheet 1
EXP-SPI-NSS1: SV3.10 ; also sheet 1
GND: J3.3 J4.3 J5.3 J6.3 J7.3 J8.3 J9.3 J10.3 SL1.16 SL2.6 SV1.6 SV2.4 SV3.2 SV4.1 SV4.11 ; also sheet 1,2,3,4,5,6,7,8
IO1: SV4.10 ; also sheet 1
IO2: SV4.9 ; also sheet 1
IO3: SV4.8 ; also sheet 1
IO4: SV4.7 ; also sheet 1
IO5: SV4.6 ; also sheet 1
IO6: SV4.5 ; also sheet 1
LCD-SPI-CS: SV1.4 ; also sheet 1
OPEN: SV3.1
SW-CLK: SV2.3 ; also sheet 1
SW-DIO: SV2.2 ; also sheet 1
USART-RX-M4: SL1.14 ; also sheet 1
USART-TX-M4: SL1.13 SV4.4 ; also sheet 1
YM1-CLK-O: SL1.1 ; also sheet 2
YM1-OUTPUT: SL1.5 ; also sheet 2
YM1-SYNC: SL1.9 ; also sheet 2
YM2-CLK-O: SL1.2 ; also sheet 3
YM2-OUTPUT: SL1.6 ; also sheet 3
YM2-SYNC: SL1.10 ; also sheet 3
YM3-CLK-O: SL1.3 ; also sheet 4
YM3-OUTPUT: SL1.7 ; also sheet 4
YM3-SYNC: SL1.11 ; also sheet 4
YM4-CLK-O: SL1.4 ; also sheet 5
YM4-OUTPUT: SL1.8 ; also sheet 5
YM4-SYNC: SL1.12 ; also sheet 5
Unconnected: SL2.5

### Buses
ADC1:3.3V,ADC-VOL-TOT,GND
ADC2:3.3V,ADC-VOL1,GND
ADC3:3.3V,ADC-VOL2,GND
ADC4:3.3V,ADC-VOL3,GND
ADC5:3.3V,ADC-VOL4,GND
ADC6:3.3V,ADC1,GND
ADC7:3.3V,ADC2,GND
ADC8:3.3V,ADC3,GND
YM-DIG-OUTPUT:5V,GND,USART-RX-M4,USART-TX-M4,YM1-CLK-O,YM1-CS,YM1-OUTPUT,YM1-SYNC,YM2-CLK-O,YM2-OUTPUT,YM2-SYNC,YM3-CLK-O,YM3-OUTPUT,YM3-SYNC,YM4-CLK-O,YM4-OUTPUT,YM4-SYNC
YM-ANA-OUTPUT:DAC-OUT-0,DAC-OUT-1,DAC-OUT-2,DAC-OUT-3,GND
LCD:5V,EXP-SPI-CLK,EXP-SPI-MISO,EXP-SPI-MOSI,GND,LCD-SPI-CS
BOOTLOADER:3.3V,GND,SW-CLK,SW-DIO

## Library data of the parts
BUT LED = con-molex:22-?-02: CONNECTOR; MF: MOLEX; OC_FARNELL: unknown; OC_NEWARK: unknown
C1-C7 C9 C10 = rcl:C-EU: CAPACITOR, European symbol; SPICEPREFIX: C
C8 C11 C12 C15-C17 C20-C22 C25-C27 C30 = +HU-Lib:100N
C13 C14 C18 C19 C23 C24 C28 C29 = +HU-Lib:10UF
C31 = +HU-Lib:0.47UF
C32 = +HU-Lib:22UF
C33-C35 C38 C39 = Clean-Kong:C-EU: CAPACITOR, European symbol
CRYSTAL2 = ABLS-3.579545MHZ-17-B-4-Y-T:ABLS-3.579545MHZ-17-B-4-Y-T
D1 = BAT20JFILM:BAT20JFILM: 23V, 1A Schottky diode, SOD-323 package; AVAILABILITY: Unavailable; DESCRIPTION: BAT20 Series Switching 1 A 0.62 V Schottky Diode Surface Mount - SOD-323; MF: STMicroelectronics; MP: BAT20JFILM; PACKAGE: SOD-323 STMicroelectronics; PRICE: None
IC1 IC4 IC7 IC10 = YM:YM3812: Dual In Line
IC2 IC5 IC8 IC11 = YM:YM3014B: Dual In Line / Socket
IC3 IC6 IC9 IC12 = linear:LM358: OP AMP also LM158; LM258; LM2904 Source: http://cache.national.com/ds/LM/LM158.pdf
IC14 = 74xx-us:74*04: Hex INVERTER; SPICEPREFIX: I
IC15 = 6N136:6N136: Vishay 6N136 DC Input, Transistor Output Optocoupler, Through-hole DIP 8 Source: Datasheet; DESCRIPTION: Vishay 6N136 DC Input, Transistor Output Optocoupler, Through-hole DIP 8; FARNELL_PART_NUMBER: 1469469; FARNELL_PRICE-STOCK: http://uk.farnell.com/jsp/displayProduct.jsp?sku=1469469&action=view; HEIGHT: 4.65mm; MANUFACTURER_NAME: Vishay; MANUFACTURER_PART_NUMBER: 6N136
J1 = LDO:CON-USB-B: USB B type connector
J2 = SparkFun-Connectors:DIN5: DIN5 Connector - Female Right Angle (frequently used as a MIDI Jack connector) This type of connector and cable is frequently used for transmitting midi data (musical instrument digital interface). It is what you usually see on a keyboard or set of electronic drums. Learn more here. For more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; PROD_ID: CONN-09481
J3-J10 = con-amp:MTA03-156: AMP connector
R1-R4 R6 R7 = +HU-Lib:1K
S1 = switch-omron:10-XX: OMRON SWITCH; MPN: B3F-1000; OC_FARNELL: 176432; OC_NEWARK: 36M3542
SL1 = con-amp-quick:M16: AMP QUICK CONNECTOR; OC_FARNELL: unknown; OC_NEWARK: unknown
SL2 = con-amp-quick:M06: AMP QUICK CONNECTOR; OC_FARNELL: unknown; OC_NEWARK: unknown
SV1 = con-amp-mt:S06P: AMP MT CONNECTOR; OC_FARNELL: unknown; OC_NEWARK: unknown
SV2 = con-lstb:MA04-1: PIN HEADER; OC_FARNELL: unknown; OC_NEWARK: unknown
SV3 = 2514-6002UB:2514-6002UB: Four-Wall Header; MPN: 2514-6002UB; OC_FARNELL: 1368928; OC_NEWARK: 46F4726; PACKAGE: Four-Wall Header, 14way; SUPPLIER: 3M
SV4 = con-lsta:FE13-1: FEMALE HEADER; OC_FARNELL: unknown; OC_NEWARK: unknown
U1 = stm32:STM32F10XRXT6: STM32F101/103 64pin LQFP
U3 = bt_regulator:LM2931: LM2931 Low Dropout Adjustable Regulator, Automotive Input voltage: 26V max 3.3V, 5V, adjustable versions Output Current in Excess of 100 mA Very Low Quiescent Current Dropout Voltage < 0.6V Reverse Battery Protection 60V Load Dump Protection −50V Reverse Transient Protection Short Circuit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
X1 = IQD-Frequency-Products:CRYSTALS-NOGND: CRYSTALS CAN NOT GROUNDED

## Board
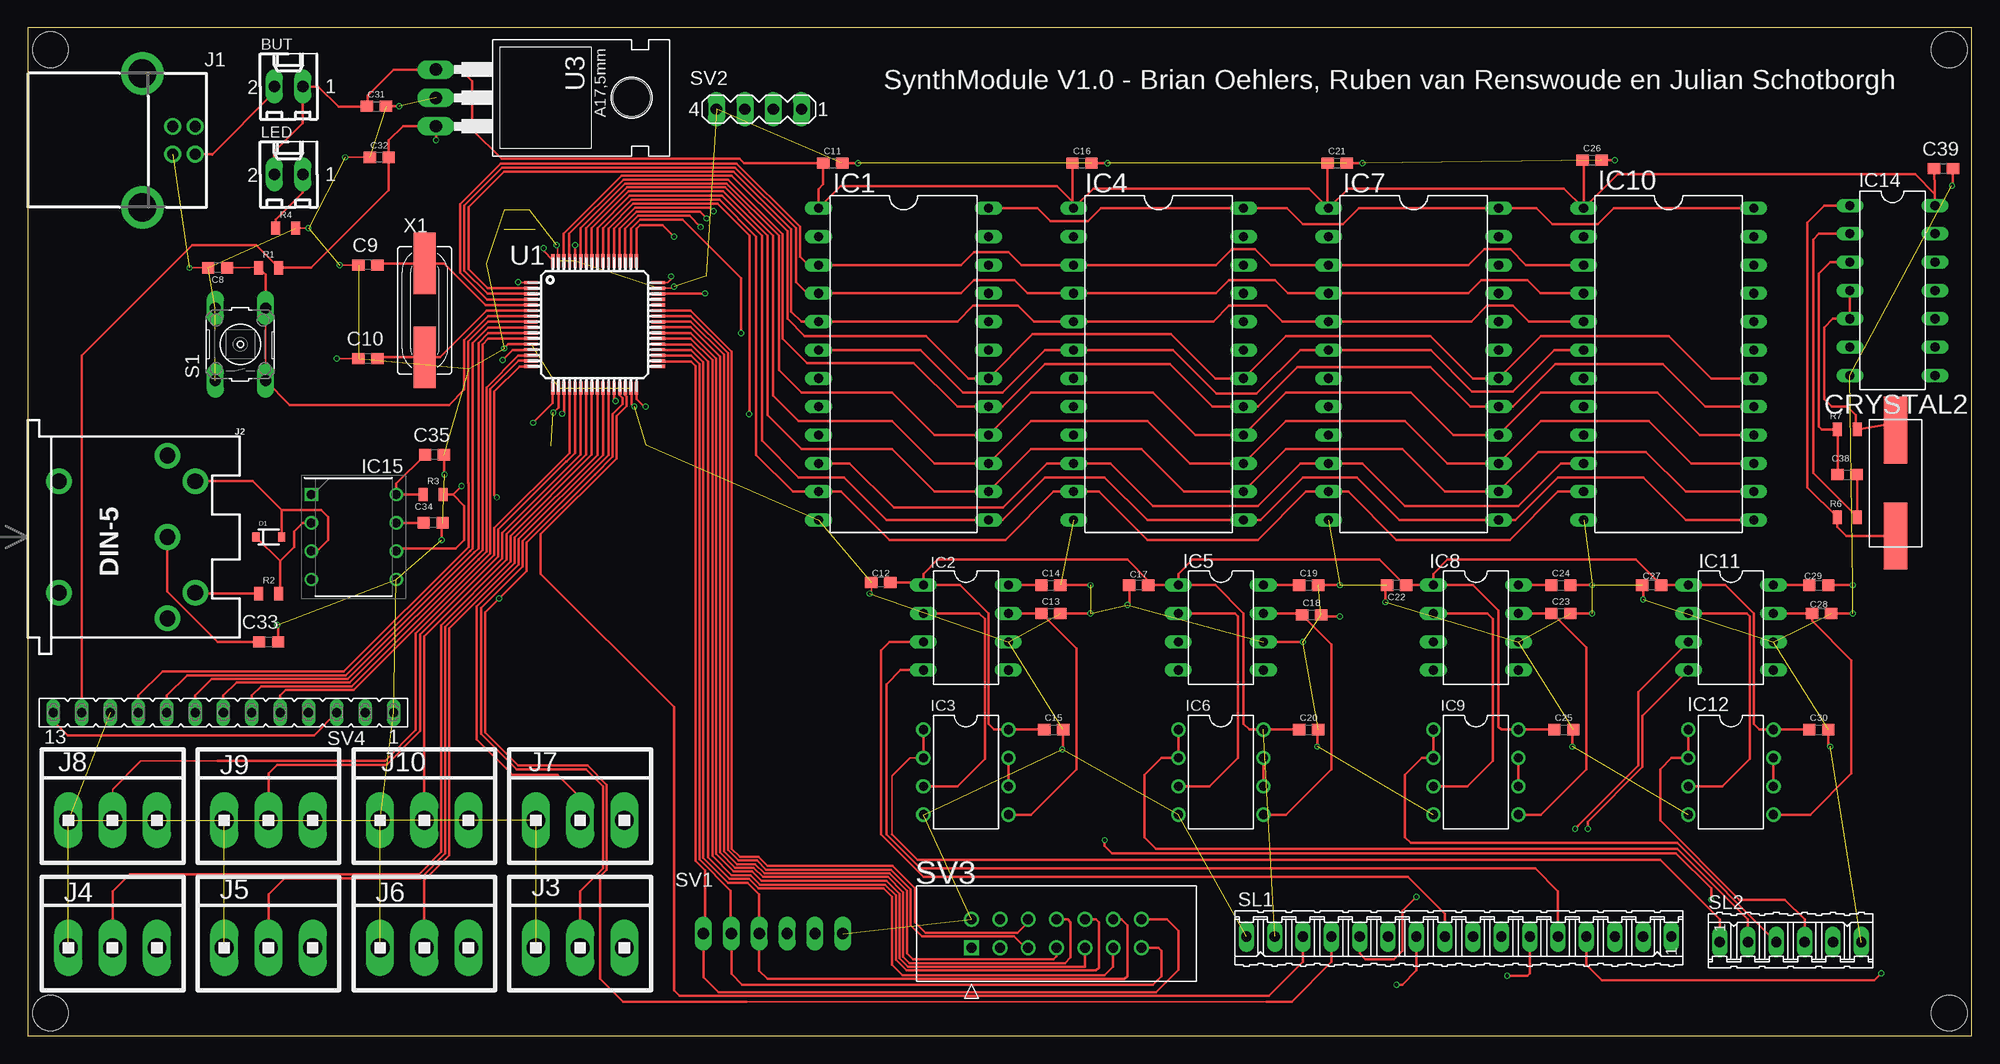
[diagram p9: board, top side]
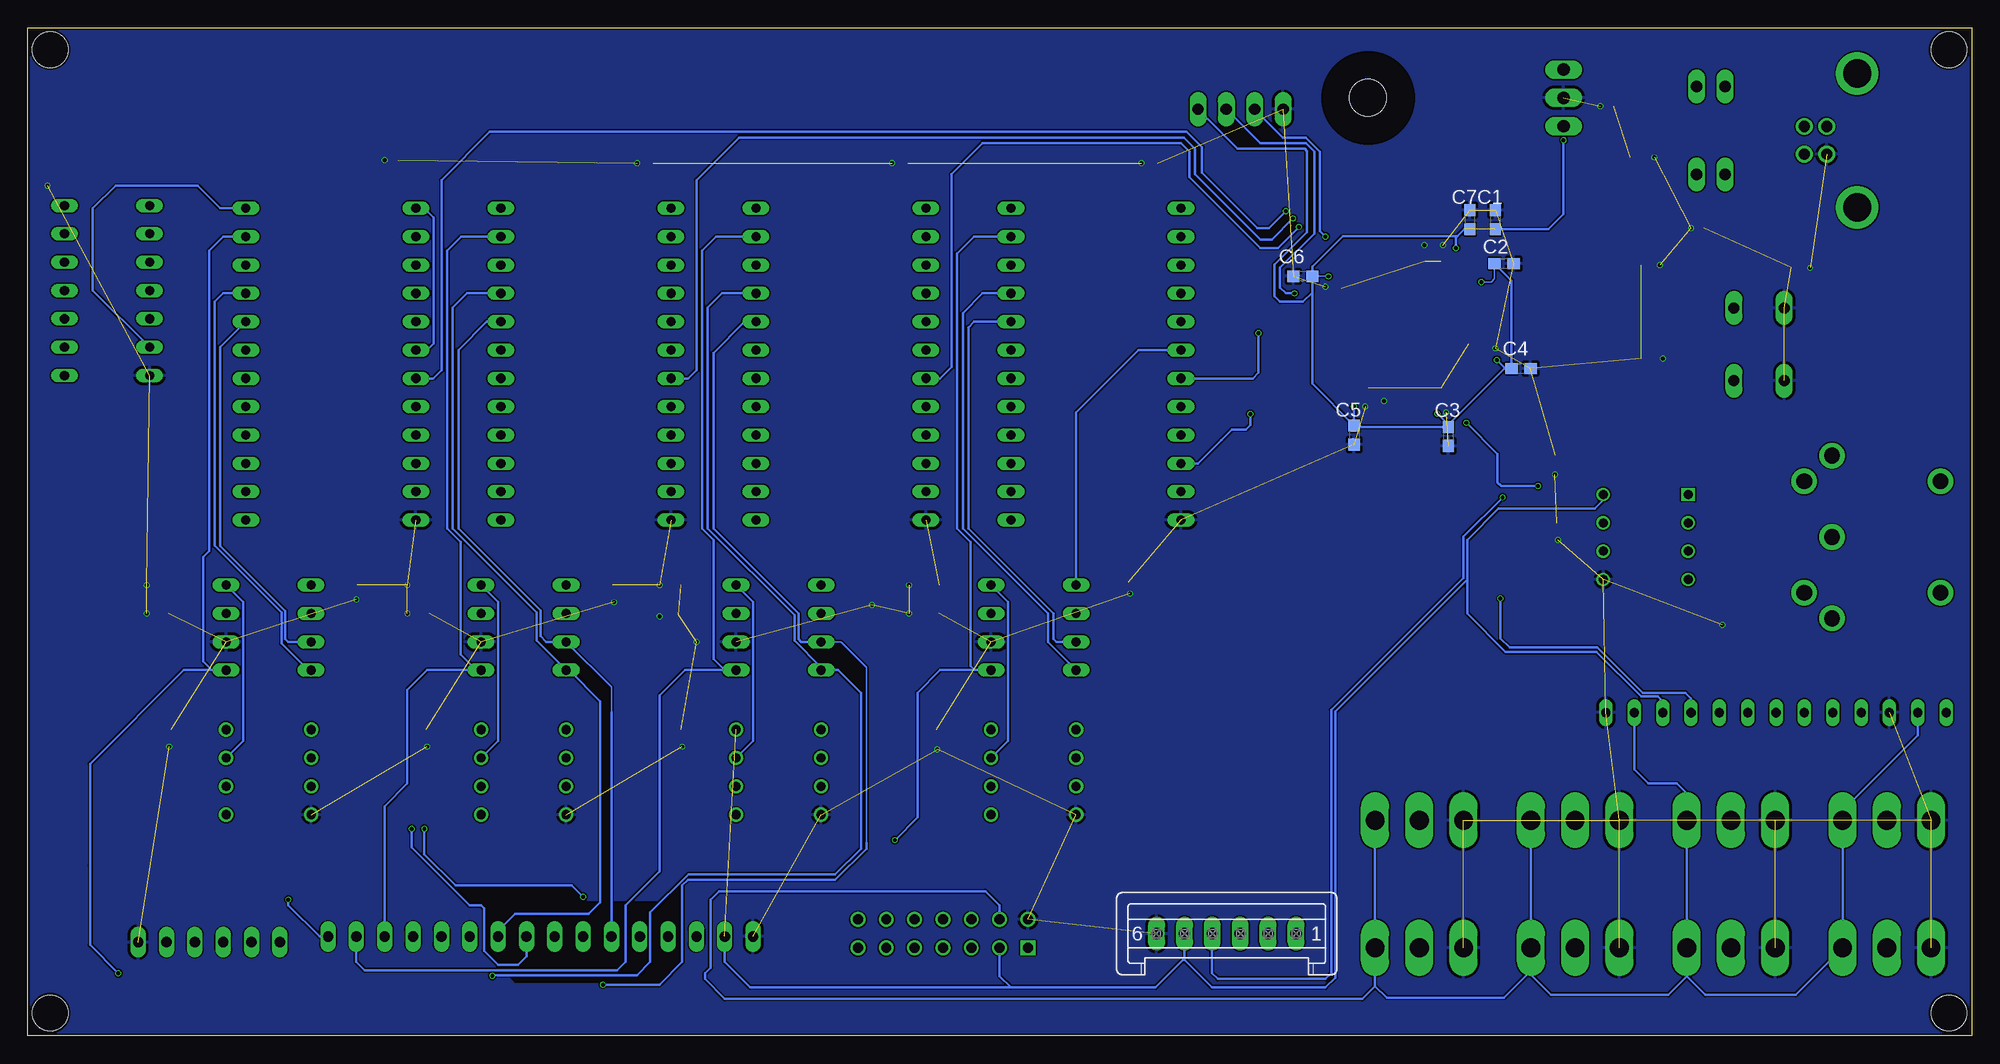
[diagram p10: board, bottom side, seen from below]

Size 174.22 x 90.35 mm. Coordinates in mm from the lower left corner, seen from the top.
Outline: 0,0 174.22,0 174.22,90.35 0,90.35 0,0
Copper layers (1*16): Top 0.035559375mm / dielectric 1.6mm / Bottom 0.035559375mm
Design rules "jlcpcb2layer": minimum track width 5mil, minimum drill 12mil, track to track 5mil, track to pad 5mil, pad to pad 5mil, via to via 5mil, smd to smd 5mil, copper to edge 8mil, drill to drill 6mil, minimum pad ring 5mil, minimum via ring 3mil, stop-mask expansion 2.5mil, vias tented up to drill 0mil, thermal gap 10mil
Holes 3.2 mm at 172.21,88.39 172.21,2.03 2.03,88.39 2.03,2.03

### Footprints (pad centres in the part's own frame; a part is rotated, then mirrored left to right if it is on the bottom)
6410-02 = drill 1.016 long: 1 1.27,0; 2 -1.27,0
C0603 = smd 1.1 x 1: 1 -0.85,0; 2 0.85,0
0603-SMD = smd 1.1 x 1: 1 -0.85,0; 2 0.85,0
ABLS-3.579545MHZ-17-B-4-Y-T-11.5X4.7X4.2 = smd 5.994 x 2.108: P$1 -4.75,0; P$2 4.75,0
SOD-323 = smd 0.63 x 0.83: A 1.15,0; C -1.15,0
YM3812 = drill 0.813 long: /CS 1.27,-7.62; /IC -8.89,-7.62; /IRQ -11.43,-7.62; /RD -1.27,-7.62; /WR -3.81,-7.62; A0 -6.35,-7.62; D0 8.89,-7.62; D1 11.43,-7.62; D2 13.97,7.62; D3 11.43,7.62; D4 8.89,7.62; D5 6.35,7.62; D6 3.81,7.62; D7 1.27,7.62; GND 13.97,-7.62; M -13.97,7.62; MO -6.35,7.62; NC@1 3.81,-7.62; NC@2 6.35,-7.62; NC@3 -1.27,7.62; NC@4 -8.89,7.62; SH -3.81,7.62; SY -11.43,7.62; VCC -13.97,-7.62
YM3014B = drill 0.813 long: BUFF -1.27,-3.81; CLK 3.81,3.81; GND 1.27,3.81; LOAD 1.27,-3.81; MP -3.81,3.81; RB -1.27,3.81; SD 3.81,-3.81; VDD -3.81,-3.81
DIL08 = drill 0.813 pad 1.27: 1 -3.81,-3.81; 2 -1.27,-3.81; 3 1.27,-3.81; 4 3.81,-3.81; 5 3.81,3.81; 6 1.27,3.81; 7 -1.27,3.81; 8 -3.81,3.81
DIL14 = drill 0.813 long: 1 -7.62,-3.81; 2 -5.08,-3.81; 3 -2.54,-3.81; 4 0,-3.81; 5 2.54,-3.81; 6 5.08,-3.81; 7 7.62,-3.81; 8 7.62,3.81; 9 5.08,3.81; 10 2.54,3.81; 11 0,3.81; 12 -2.54,3.81; 13 -5.08,3.81; 14 -7.62,3.81
DIP762W60P254L1060H465Q8N = drill 0.8 pad 1.2 square: 1 -3.81,3.81 | drill 0.8 pad 1.2: 2 -3.81,1.27; 3 -3.81,-1.27; 4 -3.81,-3.81; 5 3.81,-3.81; 6 3.81,-1.27; 7 3.81,1.27; 8 3.81,3.81
USB-B = drill 1 pad 1.508: 1 1.25,7.37; 2 -1.25,7.37; 3 -1.25,5.37; 4 1.25,5.37 | drill 2.54 pad 3.81: P$1 -6,2.63; P$2 6,2.63
DIN5-RA-PTH = drill 1.4 pad 2.286: 1 7.3,12.5; 2 0,12.5; 3 -7.3,12.5; 4 5,15; 5 -5,15; 6 -5,2.8; 7 5,2.8
1X3MTA = drill 1.676 long: 1 3.937,0; 2 -0.025,0; 3 -3.988,0
0805-SMD = smd 0.8 x 1.2: 1 -0.9,0; 2 0.9,0
B3F-10XX = drill 1.016 long: 1 -3.251,2.261; 2 3.251,2.261; 3 -3.251,-2.261; 4 3.251,-2.261
16P = drill 0.914 long: 1 -19.05,0; 2 -16.51,0; 3 -13.97,0; 4 -11.43,0; 5 -8.89,0; 6 -6.35,0; 7 -3.81,0; 8 -1.27,0; 9 1.27,0; 10 3.81,0; 11 6.35,0; 12 8.89,0; 13 11.43,0; 14 13.97,0; 15 16.51,0; 16 19.05,0
06P = drill 0.914 long: 1 -6.35,0; 2 -3.81,0; 3 -1.27,0; 4 1.27,0; 5 3.81,0; 6 6.35,0
S06P = drill 1.016 long: 1 6.25,0; 2 3.75,0; 3 1.25,0; 4 -1.25,0; 5 -3.75,0; 6 -6.25,0
MA04-1 = drill 1.016 long: 1 -3.81,0; 2 -1.27,0; 3 1.27,0; 4 3.81,0
3M_2514-6002UB = drill 0.889 square: 1 0,2.54 | drill 0.889: 2 0,0; 3 -2.54,2.54; 4 -2.54,0; 5 -5.08,2.54; 6 -5.08,0; 7 -7.62,2.54; 8 -7.62,0; 9 -10.16,2.54; 10 -10.16,0; 11 -12.7,2.54; 12 -12.7,0; 13 -15.24,2.54; 14 -15.24,0
FE13 = drill 0.813 long: 1 -15.24,0; 2 -12.7,0; 3 -10.16,0; 4 -7.62,0; 5 -5.08,0; 6 -2.54,0; 7 0,0; 8 2.54,0; 9 5.08,0; 10 7.62,0; 11 10.16,0; 12 12.7,0; 13 15.24,0
TQFP64 = smd 1.2 x 0.3: 1 -5.7,3.75; 2 -5.7,3.25; 3 -5.7,2.75; 4 -5.7,2.25; 5 -5.7,1.75; 6 -5.7,1.25; 7 -5.7,0.75; 8 -5.7,0.25; 9 -5.7,-0.25; 10 -5.7,-0.75; 11 -5.7,-1.25; 12 -5.7,-1.75; 13 -5.7,-2.25; 14 -5.7,-2.75; 15 -5.7,-3.25; 16 -5.7,-3.75; 33 5.7,-3.75; 34 5.7,-3.25; 35 5.7,-2.75; 36 5.7,-2.25; 37 5.7,-1.75; 38 5.7,-1.25; 39 5.7,-0.75; 40 5.7,-0.25; 41 5.7,0.25; 42 5.7,0.75; 43 5.7,1.25; 44 5.7,1.75; 45 5.7,2.25; 46 5.7,2.75; 47 5.7,3.25; 48 5.7,3.75 | smd 0.3 x 1.2: 17 -3.75,-5.7; 18 -3.25,-5.7; 19 -2.75,-5.7; 20 -2.25,-5.7; 21 -1.75,-5.7; 22 -1.25,-5.7; 23 -0.75,-5.7; 24 -0.25,-5.7; 25 0.25,-5.7; 26 0.75,-5.7; 27 1.25,-5.7; 28 1.75,-5.7; 29 2.25,-5.7; 30 2.75,-5.7; 31 3.25,-5.7; 32 3.75,-5.7; 49 3.75,5.7; 50 3.25,5.7; 51 2.75,5.7; 52 2.25,5.7; 53 1.75,5.7; 54 1.25,5.7; 55 0.75,5.7; 56 0.25,5.7; 57 -0.25,5.7; 58 -0.75,5.7; 59 -1.25,5.7; 60 -1.75,5.7; 61 -2.25,5.7; 62 -2.75,5.7; 63 -3.25,5.7; 64 -3.75,5.7
TO220BH = drill 1.118 long: 1 -2.54,-6.35; 2 0,-6.35; 3 2.54,-6.35 | hole 3.302: 0,11.176
HC49-4-HSMX = smd 5.5 x 2: 1 -4.2,0; 2 4.2,0

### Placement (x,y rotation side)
BUT  23.37,85.09 0 top
C1  42.67,73.15 90 bottom
C2  41.91,69.22 0 bottom
C3  46.91,53.72 270 bottom
C4  40.39,59.82 0 bottom
C5  55.35,53.85 270 bottom
C6  59.94,68.07 180 bottom
C7  44.96,73.15 90 bottom
C8  17.02,68.83 180 top
C9  30.48,69.09 180 top
C10  30.48,60.71 180 top
C11  72.14,78.23 0 top
C12  76.45,40.64 180 top
C13  91.69,37.85 0 top
C14  91.69,40.39 0 top
C15  91.95,27.43 0 top
C16  94.49,78.23 0 top
C17  99.57,40.39 180 top
C18  115.06,37.72 0 top
C19  114.81,40.39 0 top
C20  114.81,27.43 0 top
C21  117.35,78.23 0 top
C22  122.68,40.39 180 top
C23  137.41,37.85 0 top
C24  137.41,40.39 0 top
C25  137.67,27.43 0 top
C26  140.21,78.49 0 top
C27  145.54,40.39 180 top
C28  160.78,37.85 0 top
C29  160.53,40.39 0 top
C30  160.53,27.43 0 top
C31  31.24,83.31 0 top
C32  31.5,78.74 180 top
C33  21.59,35.31 0 top
C34  36.32,45.97 180 top
C35  36.45,52.07 180 top
C38  163.07,50.29 0 top
C39  171.7,77.72 180 top
CRYSTAL2  167.39,49.53 270 top
D1  21.59,44.7 0 top
IC1  78.49,60.2 270 top
IC2  84.07,36.58 270 top
IC3  84.07,23.62 270 top
IC4  101.35,60.2 270 top
IC5  106.93,36.58 270 top
IC6  106.93,23.62 270 top
IC7  124.21,60.2 270 top
IC8  129.79,36.58 270 top
IC9  129.79,23.62 270 top
IC10  147.07,60.2 270 top
IC11  152.65,36.58 270 top
IC12  152.65,23.62 270 top
IC14  167.13,66.8 270 top
IC15  29.21,44.7 0 top
J1  7.62,80.26 270 top
J2  0,44.7 270 top
J3  49.53,7.87 0 top
J4  7.62,7.87 0 top
J5  21.59,7.87 0 top
J6  35.56,7.87 0 top
J7  49.53,19.3 0 top
J8  7.62,19.3 0 top
J9  21.59,19.3 0 top
J10  35.56,19.3 0 top
LED  23.37,77.22 0 top
R1  21.59,68.83 0 top
R2  21.59,39.62 0 top
R3  36.32,48.51 0 top
R4  23.11,72.39 0 top
R6  163.07,46.48 180 top
R7  163.07,54.36 0 top
S1  19.05,61.98 90 top
SL1  128.27,8.89 180 top
SL2  157.99,8.38 0 top
SV1  66.8,9.14 0 bottom
SV2  65.53,83.06 180 top
SV3  84.58,10.41 180 top
SV4  17.53,28.96 180 top
U1  50.8,63.75 0 top
U3  42.93,84.07 270 top
X1  35.56,65.02 270 top

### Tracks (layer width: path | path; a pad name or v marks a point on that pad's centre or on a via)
3.3V  (via drill 0.35)  (1 unrouted)
  Top 0.152: U1.48 57.34,67.5 57.66,67.82 v57.66,68.07 | U1.64 47.05,69.54 | U1.1 44.26,67.5 44.2,67.56 v43.94,67.56
  Top 0.203: U1.13 45.06,61.47 43.43,61.47 v42.55,60.58 | 47.05,69.54 46.23,70.36 v46.23,70.61 | SV4.12 4.83,60.96 14.73,70.87 20.46,70.87 R1.2 25.4,68.83 32.35,75.78 C32.1 32.35,80.26 33.62,81.53 U3.3 v36.58,80.26 | U1.32 54.55,57.08 55.24,56.39 v55.37,56.39 | U1.19 48.05,55.92 v47.88,55.75
  Bottom 0.152: 55.37,55.23 55.37,54.72 | v57.66,68.07 C6.1 59.18,68.16 | C2.1 42.76,67.86 43.05,67.56 v43.94,67.56
  Bottom 0.203: C2.1 41.24,67.69 C4.1 41.78,59.82 | 41.78,59.82 41.87,59.82 46.91,54.77 C3.1 | 25.53,5.31 23.88,3.66 15.77,3.66 J4.1 J8.1 11.56,20.19 4.83,26.92 SV4.12 | 25.53,5.31 J5.1 J9.1 25.53,21.72 26.42,22.61 28.96,22.61 30.23,23.88 SV4.2 | 25.53,5.31 27.18,3.66 37.69,3.66 39.5,5.46 39.5,5.82 | 39.5,5.82 41.91,3.4 52.43,3.4 53.47,4.45 | 53.47,4.45 J3.1 J7.1 | v46.23,70.61 46.23,71.54 46.1,71.67 | C7.1 45.47,72.3 46.1,71.67 | J10.1 J6.1 39.5,5.82 | 53.47,4.45 54.61,3.3 111.76,3.3 113.54,5.08 113.54,5.59 113.03,6.1 113.03,12.19 112.27,12.95 88.39,12.95 87.12,11.68 SV3.4 | C6.1 59.09,66.64 59.94,65.79 61.98,65.79 62.48,66.29 62.48,69.12 59.56,72.04 59.56,79.31 59.76,79.5 65.79,79.5 SV2.1 | C1.1 37.93,72.3 36.58,73.66 v36.58,80.26 | C3.1 54.71,54.57 54.84,54.7 | 54.84,54.7 C5.1 | 54.84,54.7 55.37,55.23 | v55.37,56.39 55.37,54.72 C5.1 | C5.1 59.09,58.45 C6.1 | C6.1 59.09,68.92 56.35,71.67 46.1,71.67 | v47.88,55.75 46.91,54.79 C3.1 | v42.55,60.58 41.78,59.82
5V  (1 unrouted)
  Top 0.152: 30.61,83.1 30.44,83.27 C31.1 30.39,83.73
  Top 0.203: C35.2 33.02,49.49 IC15.8 R3.1 | 93.64,74.76 93.64,74.26 IC4.VCC 95.5,75.95 114.81,75.95 IC7.VCC | 93.64,74.76 C16.1 | IC7.VCC 116.5,74.26 C21.1 | IC10.VCC 139.45,78.4 C26.1 | 93.64,74.76 92.24,76.16 72.86,76.16 IC1.VCC 70.87,75.91 71.29,76.33 C11.1 64.17,78.23 63.79,78.61 42.44,78.61 39.83,81.23 39.83,85.55 38.76,86.61 U3.1 32.77,86.61 30.44,84.28 30.44,83.27 27.86,83.27 26.04,85.09 BUT.1 24.64,81.79 22.1,79.25 LED.2 | IC7.VCC 118.36,75.95 137.67,75.95 IC10.VCC | IC1./RD 80.01,61.47 83.82,57.66 87.38,57.66 91.19,61.47 IC4./RD 102.62,61.47 106.53,57.56 110.13,57.56 114.05,61.47 IC7./RD 125.73,61.47 129.44,57.76 133.12,57.76 136.83,61.47 IC10./RD | C39.2 170.94,76.37 IC14.14 170.94,75.44 169.16,77.22 142.49,77.22 IC10.VCC | C12.1 80.01,40.64 IC2.VDD | C15.1 IC3.8 86.61,27.43 86.11,27.94 86.11,37.85 83.57,40.39 IC2.VDD | IC5.VDD C17.1 100.42,40.81 98.55,42.67 81.53,42.67 80.26,41.4 IC2.VDD | IC5.VDD 106.43,40.39 108.97,37.85 108.97,27.94 109.47,27.43 IC6.8 C20.1 | IC5.VDD 103.12,41.4 104.39,42.67 121.16,42.67 123.44,40.39 C22.1 IC8.VDD | IC8.VDD 129.54,40.39 131.83,38.1 131.83,27.69 132.08,27.43 IC9.8 C25.1 | IC8.VDD 125.98,41.4 127.25,42.67 144.11,42.67 C27.1 IC11.VDD 152.15,40.39 154.69,37.85 154.69,27.94 155.19,27.43 IC12.8 C30.1 | SV4.13 2.29,28.19 3.56,26.92 25.65,26.92 SV4.3
  Bottom 0.203: 45.21,40.89 45.21,41.27 45.21,44.45 42.42,47.24 33.78,47.24 33.02,48.01 IC15.8 | 45.21,40.89 45.21,37.85 41.78,34.42 33.61,34.42 29.6,30.4 28.12,30.4 27.69,29.97 SV4.3 | IC10./RD 138.43,61.47 137.87,62.03 137.87,73.36 138.68,74.17 IC10.VCC | IC1./RD 74.68,61.47 80.26,55.88 IC2.VDD | 70.55,6.8 68.07,4.32 57.91,4.32 57.02,5.21 57.02,29.08 45.21,40.89 | SV1.5 70.55,6.8 | 70.55,6.8 70.67,6.8 73.15,4.32 86.11,4.32 | 86.11,4.32 109.47,4.32 111.76,6.6 SL1.15 | SV3.3 87.12,5.33 86.11,4.32
5VBUTTON
  Top 0.203: J1.1 16.49,79.01 16.51,78.99 22.1,84.58 BUT.2
ADC1
  Top 0.152: 17.02,24.64 10.13,24.64 7.59,22.1 J8.2
  Top 0.203: U1.20 48.55,52.25 41.81,45.51 41.81,43.08 34.77,36.04 34.77,27.4 32,24.64 17.02,24.64
ADC2
  Top 0.203: U1.21 49.05,52.23 48.28,51.46 48.26,51.46 42.16,45.36 42.16,42.94 35.17,35.95 35.17,27.3 32.15,24.28 22.35,24.28 21.57,23.5 J9.2
ADC3
  Top 0.203: U1.22 49.55,52.09 42.52,45.06 42.52,42.79 35.53,35.8 35.53,22.13 35.53,22.12 J10.2
ADC-VOL1
  Top 0.203: U1.23 50.05,52.08 42.93,44.96 42.93,42.67 37.05,36.79 37.05,16.47 35.05,14.48 9.14,14.48 7.59,12.93 J4.2
ADC-VOL2
  Top 0.203: U1.24 50.55,52.08 43.28,44.81 43.28,42.52 37.4,36.64 37.4,16.32 35.2,14.12 23.01,14.12 21.57,12.68 J5.2
ADC-VOL3
  Top 0.203: U1.25 51.05,52.07 43.64,44.65 43.64,42.37 37.76,36.49 37.76,16.17 35.53,13.95 J6.2
ADC-VOL4
  Top 0.203: U1.26 51.55,52.06 43.99,44.51 43.99,42.23 40.24,38.47 40.24,26.57 43.44,23.37 47.5,23.37 49.51,21.36 J7.2
ADC-VOL-TOT
  Top 0.203: U1.27 52.05,52.05 44.35,44.35 44.35,42.06 40.64,38.35 40.64,27.04 43.8,23.88 50.04,23.88 51.56,22.35 51.56,14.99 49.51,12.93 J3.2
DAC-OUT-0
  Top 0.152: IC3.2 79.08,24.89 77.47,23.28 77.47,18.03
  Top 0.203: IC3.1 IC3.2 | SL2.1 151.64,10.41 146.3,15.75 79.76,15.75 77.47,18.03
DAC-OUT-1
  Top 0.203: IC6.1 IC6.2 101.6,24.89 100.08,23.37 100.08,17.78 101.09,16.76 147.83,16.76 154.18,10.41 SL2.2
DAC-OUT-2
  Top 0.203: IC9.1 IC9.2 124.97,24.89 123.44,23.37 123.44,17.78 123.95,17.27 147.83,17.27 SL2.3
DAC-OUT-3
  Top 0.203: IC12.1 IC12.2 147.32,24.89 146.3,23.88 146.3,19.3 153.42,12.19 157.48,12.19 159.26,10.41 SL2.4
EXP1-INTA
  Top 0.203: U1.40 59.41,63.5 62.03,60.89 62.03,16.42 63.41,15.04 65.06,15.04 65.88,14.22 77.09,14.22 78.46,12.86 78.46,7.05 79.01,6.5 92.96,6.5 93.47,7.01 93.47,10.16 93.22,10.41 SV3.8
EXP1-INTB
  Top 0.203: U1.41 59.41,64 62.38,61.04 62.38,16.53 63.55,15.37 65.2,15.37 66.01,14.55 77.23,14.55 78.79,12.99 78.79,7.37 79.32,6.83 91.92,6.83 92.2,7.11 SV3.7
EXP2-INTA
  Top 0.203: U1.42 59.42,64.5 62.74,61.18 62.74,16.64 63.68,15.7 65.34,15.7 66.15,14.88 77.37,14.88 79.12,13.13 79.12,9.91 80.14,8.89 88.39,8.89 89.41,7.87 SV3.5
EXP2-INTB
  Top 0.203: U1.43 59.42,65 63.09,61.33 63.09,16.75 63.82,16.03 65.47,16.03 66.29,15.21 77.5,15.21 79.5,13.22 79.5,10.16 80.44,9.22 88.72,9.22 89.66,10.16 SV3.6
EXP-RST
  Top 0.203: U1.39 59.41,63 61.7,60.72 61.7,16.28 63.27,14.71 64.93,14.71 65.77,13.87 76.98,13.87 78.13,12.72 78.13,6.92 78.88,6.17 94.74,6.17 SV3.9
EXP-SPI-CLK
  Top 0.203: U1.34 56.55,60.45 59.44,60.45 59.87,60.02 59.87,15.65 60.71,14.81 60.71,9.3 SV1.1 60.55,5.23 61.9,3.89 101.09,3.89 103.12,5.92 103.12,9.4 102.11,10.41 SV3.14
EXP-SPI-MISO
  Top 0.203: U1.35 56.54,60.96 59.44,60.96 60.2,60.2 60.2,15.79 62.99,12.99 62.99,9.2 SV1.2 63.05,5.53 64.01,4.57 100.84,4.57 101.6,5.33 101.6,7.62 101.35,7.87 SV3.13
EXP-SPI-MOSI
  Top 0.203: U1.36 56.54,61.47 59.44,61.47 60.53,60.38 60.53,15.93 62.74,13.72 64.52,13.72 65.55,12.68 SV1.3 65.55,5.82 66.29,5.08 98.3,5.08 98.55,5.33 98.55,9.91 98.04,10.41 SV3.12
EXP-SPI-NSS0
  Top 0.203: U1.37 56.53,61.98 59.43,61.98 60.96,60.45 60.96,16 62.92,14.05 64.65,14.05 65.49,13.21 76.71,13.21 77.47,12.45 77.47,6.35 78.41,5.41 96.52,5.41 97.28,6.17 SV3.11
EXP-SPI-NSS1
  Top 0.203: U1.38 59.41,62.5 61.37,60.54 61.37,16.1 63.09,14.38 64.79,14.38 65.63,13.54 76.84,13.54 77.8,12.58 77.8,6.78 78.74,5.84 95.76,5.84 96.01,6.1 96.01,10.16 95.76,10.41 SV3.10
GND  (via drill 0.35)  (76 unrouted)
  Top 0.152: U1.47 57.75,67 v57.91,67.16 | U1.63 47.5,69.51 47.5,70.87 v47.39,70.87 | C32.2 v28.45,78.74 | v14.48,68.83 C8.2 | C10.2 v27.69,60.71 | C9.2 v27.94,69.09 | C12.2 75.6,39.79 v75.44,39.62 | R4.2 v25.15,72.39
  Top 0.203: v37.34,50.29 37.3,50.33 C35.1 | v22.35,36.83 22.44,36.74 C33.2 | C34.1 37.08,45.89 v37.08,44.45 | U1.18 47.55,56.31 v47.1,55.86 v47.1,55.85 | U1.28 52.55,57.03 v52.68,56.9 | U1.31 54.1,58 54.1,56.64 v54.36,56.39 | v49.05,70.87 v49.05,70.86 U1.60 | C15.2 92.8,25.74 v92.71,25.65 | C17.2 98.72,38.77 v98.55,38.61 | C20.2 115.57,27.34 v115.57,25.91 | C14.2 v95.25,40.39 | C13.2 v95.25,37.85 | C19.2 v117.6,40.39 | v117.6,37.59 116.04,37.59 C18.2 | C24.2 v140.21,40.39 | C23.2 v140.21,37.85 | C25.2 138.43,27.34 v138.43,25.91 | C30.2 161.38,26.07 v161.54,25.91 | C11.2 v74.42,78.23 | C16.2 v96.77,78.23 | C21.2 v119.63,78.23 | C26.2 v142.24,78.49 | C39.1 172.55,76.29 v172.47,76.2 | C29.2 v163.58,40.39 | C28.2 v163.58,37.85 | C22.2 121.67,40.22 v121.67,38.86 | IC5.GND v114.3,35.31 | C27.2 144.78,40.3 v144.78,39.12 | C31.2 v33.27,83.31 | U1.12 43.06,62 v42.67,61.62
  pour Bottom: -0.25,90.93 174.5,90.93 175.51,89.92 175.51,0.51 172.72,-2.29 1.27,-2.29 -5.08,4.06 -5.08,86.11
  cutout Bottom: 115.82,13.21 117.09,11.94 133.35,11.94 133.35,7.62 130.56,4.83 117.6,4.83 115.82,6.6
IO1
  Top 0.203: U1.8 41.27,64 39.47,62.2 39.47,49.56 39.49,49.54 39.49,43.81 28.32,32.64 12.06,32.64 9.91,30.48 SV4.10
IO2
  Top 0.203: U1.9 41.27,63.5 39.88,62.1 39.88,43.69 39.62,43.43 28.49,32.31 14.28,32.31 12.45,30.48 SV4.9
IO3
  Top 0.203: U1.10 45.09,62.99 41.27,62.99 40.39,62.1 40.39,43.69 40.01,43.31 40,43.31 28.67,31.98 16.48,31.98 14.99,30.48 SV4.8
IO4
  Top 0.203: U1.11 45.08,62.48 41.25,62.48 40.74,61.98 40.74,43.54 28.85,31.65 18.69,31.65 17.53,30.48 SV4.7
IO5
  Top 0.203: U1.14 45.06,60.96 43.94,60.96 41.1,58.12 41.1,43.38 40.39,42.67 40.38,42.67 29.03,31.32 20.9,31.32 20.07,30.48 SV4.6
IO6
  Top 0.203: U1.15 43.99,60.5 41.45,57.96 41.45,43.23 29.21,30.99 23.11,30.99 22.61,30.48 SV4.5
LCD-SPI-CS  (via drill 0.35)
  Top 0.203: U1.16 44.08,60 41.81,57.73 41.81,48.49 v42.04,48.26
  Bottom 0.203: v42.04,48.26 45.57,44.73 45.57,41.05 57.4,29.21 57.4,5.59 57.91,5.08 67.56,5.08 68.07,5.59 68.07,9.12 SV1.4
N$1
  Top 0.152: C9.1 31.35,69.11
  Top 0.203: U1.5 41.05,65.5 37.33,69.22 X1.1 31.47,69.22 31.35,69.11
N$2
  Top 0.152: C10.1 31.41,60.79
  Top 0.203: U1.6 41.13,65 36.95,60.82 X1.2 31.45,60.82 31.41,60.79
N$3
  Top 0.203: IC2.BUFF 85.27,37.85 85.78,37.34 85.78,24.82 83.31,22.35 IC3.3
N$4
  Top 0.203: IC5.RB 114.08,37.85 C18.1 116.84,35.09 116.84,23.88 112.78,19.81 IC6.5
N$5
  Top 0.203: IC2.MP C14.1 | IC3.7 IC3.6
  Bottom 0.203: IC2.MP 86.36,38.86 86.36,26.42 IC3.7
N$6
  Top 0.203: IC5.BUFF 108.2,37.85 108.46,37.59 108.46,24.89 105.92,22.35 IC6.3
N$7
  Top 0.203: IC8.RB C23.1 136.65,37.85 139.7,34.8 139.7,23.88 135.64,19.81 IC9.5
N$8
  Top 0.203: IC5.MP C19.1 | IC6.6 IC6.7
  Bottom 0.203: IC5.MP 109.22,38.86 109.22,26.42 IC6.7
N$9
  Top 0.203: IC9.3 129.03,22.35 131.32,24.64 131.32,37.34 130.81,37.85 IC8.BUFF
N$10
  Top 0.203: IC11.RB C28.1 159.93,37.17 163.45,33.66 163.45,23.5 159.77,19.81 IC12.5
N$11
  Top 0.203: IC8.MP C24.1 | IC9.7 IC9.6
  Bottom 0.203: IC8.MP 132.08,38.86 132.08,26.42 IC9.7
N$12
  Top 0.203: IC11.BUFF 154.08,37.85 154.33,37.59 154.33,24.79 151.89,22.35 IC12.3
N$13
  Top 0.152: 22.1,72.51 R4.1
  Top 0.203: R4.1 22.21,73.14 24.64,75.56 LED.1
N$14
  Top 0.203: C29.1 IC11.MP | IC12.6 IC12.7
  Bottom 0.203: IC11.MP 154.94,38.86 154.94,26.42 IC12.7
N$15
  Top 0.203: IC2.RB C13.1 93.98,34.71 93.98,23.88 89.92,19.81 IC3.5
N$16
  Top 0.203: J2.5 20.15,49.7 22.73,47.12 | D1.A 22.74,47.11 22.73,47.12 | 22.73,47.12 26.29,47.12 26.92,46.48 26.92,44.45 25.91,43.43 IC15.3
N$17
  Top 0.203: D1.C 22.61,42.54 | R2.2 22.61,39.74 22.61,42.54 | 22.61,42.54 23.88,43.81 23.88,45.21 24.64,45.97 IC15.2
N$18
  Top 0.203: J2.2 12.5,39.82 17.02,35.31 C33.1
N$19
  Top 0.203: R2.1 15.08,39.62 J2.4
N$20
  Top 0.203: CRYSTAL2.P$1 166.85,54.82 R7.2 163.83,54.49 163.83,55.63 163.07,56.39 161.7,56.39 161.04,57.05 161.04,63.5 161.8,64.26 IC14.5 IC14.4
N$21
  Top 0.203: C34.2 IC15.7
N$25
  Top 0.203: IC14.2 160.53,71.88 160.02,71.37 160.02,50.43 R6.1 163.97,50.24 C38.2
N$26
  Top 0.152: 162.22,54.31 R7.1
  Top 0.203: IC14.3 161.54,69.34 160.53,68.33 160.53,54.61 160.78,54.36 R7.1 | C38.1 162.22,54.31
N$27
  Top 0.203: IC14.1 161.04,74.42 159.51,72.9 159.51,49.14 R6.2 162.17,45.6 162.99,44.78 CRYSTAL2.P$2
RST
  Top 0.152: C8.1 19.93,68.83 20.63,68.89 R1.1 | S1.3 S1.4
  Top 0.203: U1.7 41.26,64.5 39.12,62.36 39.12,57.91 37.75,56.55 23.48,56.55 S1.3 | R1.1 21.31,68.21 S1.4
SW-CLK  (via drill 0.35)
  Top 0.203: U1.49 54.55,72.33 54.86,72.64 56.9,72.64 v57.91,71.63
  Bottom 0.203: v57.91,71.63 58.42,72.14 58.42,79.25 59.69,80.52 61.09,80.52 | SV2.3 61.72,80.52 61.09,80.52 | 61.09,80.52
SW-DIO  (via drill 0.35)
  Top 0.203: v60.71,66.55 60.66,66.5 U1.46
  Bottom 0.203: v60.71,66.55 61.47,66.55 61.98,67.06 61.98,68.83 58.93,71.88 58.93,79.25 59.69,80.01 63.75,80.01 SV2.2
USART-RX-M4
  Top 0.203: U1.30 53.55,57.42 53.67,57.3 53.67,56.46 52.76,55.55 52.76,51.74 45.97,44.96 45.97,41.4 57.91,29.46 57.91,4.06 58.42,3.56 111.25,3.56 114.3,6.6 SL1.14
USART-RX-MIDI  (via drill 0.35)
  Top 0.203: 38.1,48.51 R3.2 | IC15.6 33.27,43.69 38.35,43.69 39.12,44.45 39.12,47.5 38.1,48.51 | v38.86,49.28 38.1,48.51 | v45.29,54.94 47.05,56.7 U1.17
  Bottom 0.203: v45.29,54.94 42.5,52.15 42.5,49.61 42.16,49.28 v38.86,49.28
USART-TX-M4  (via drill 0.35)
  Top 0.152: 64.41,3.05 111,3.05
  Top 0.203: U1.29 53.05,57.42 53.31,57.16 53.31,56.63 52.41,55.73 52.41,51.9 50.82,50.32 50.82,50.31 44.7,44.2 44.7,41.65 v42.23,39.18 40.97,37.92 40.97,27.18 43.94,24.21 50.17,24.21 51.89,22.49 51.89,14.85 51.31,14.27 51.31,5.08 53.34,3.05 64.41,3.05 | 111,3.05 113.28,3.05 116.84,6.6 SL1.13
  Bottom 0.203: SV4.4 25.15,30.23 25.65,30.73 29.46,30.73 33.53,34.8 41.41,34.8 42.23,35.62 v42.23,39.18
YM1-CLK-O  (via drill 0.35)
  Top 0.203: v96.52,17.53 96.52,17.02 97.18,16.36 147.73,16.36 150.88,13.21 v150.88,12.19
  Bottom 0.203: IC1.SY 89.41,71.63 90.93,70.1 90.93,45.47 89.71,44.25 89.71,33.15 89.33,32.77 IC2.CLK 92.46,32.77 94.49,30.73 94.49,19.56 v96.52,17.53 | v150.88,12.19 150.88,11.68 148.08,8.89 SL1.1
YM1-CS  (via drill 0.35)
  Top 0.203: U1.50 54.05,72.34 54.86,73.15 58.67,73.15 63.93,67.9 v63.93,62.99
  Bottom 0.203: v63.93,62.99 63.93,59.44 64.44,58.93 IC1./CS
YM1-OUTPUT
  Top 0.203: IC2.SD 78.23,32.77 76.96,31.5 76.96,18.03 80.01,14.99 135.13,14.99 137.16,12.95 SL1.5
  Bottom 0.203: IC1.MO 88.65,66.55 90.42,64.77 90.42,45.47 82.8,37.85 82.8,35.31 IC2.SD
YM1-SYNC
  Top 0.203: IC2.LOAD 77.22,35.31 76.45,34.54 76.45,18.03 80.26,14.22 123.7,14.22 127,10.92 SL1.9
  Bottom 0.203: IC1.SH 89.41,64.01 89.92,63.5 89.92,45.47 82.3,37.85 82.3,35.56 82.04,35.31 IC2.LOAD
YM2-CLK-O
  Bottom 0.203: IC4.SY 112.52,71.63 113.79,70.36 113.79,45.47 112.78,44.45 112.78,33.78 111.76,32.77 IC5.CLK 115.32,32.77 117.6,30.48 117.6,14.73 120.65,11.68 120.65,6.6 121.41,5.84 144.02,5.84 144.78,6.6 SL1.2
YM2-CS  (via drill 0.35)
  Top 0.203: U1.51 53.55,72.35 54.71,73.51 59.3,73.51 v60.31,72.5
  Bottom 0.203: v60.31,72.5 62.2,70.61 63.75,70.61 70.1,76.96 70.1,79.25 70.87,80.01 88.65,80.01 91.44,77.22 91.44,59.94 92.46,58.93 IC4./CS
YM2-OUTPUT  (via drill 0.35)
  Top 0.203: v132.59,5.35 134.38,5.35 134.62,5.59 SL1.6
  Bottom 0.203: IC4.MO 112.01,66.55 113.28,65.28 113.28,45.47 105.51,37.69 105.51,35.41 103.12,33.02 IC5.SD 101.6,32.77 99.57,30.73 99.57,16.76 101.85,14.48 115.02,14.48 118.44,11.06 118.44,6.6 119.62,5.43 132.51,5.43 v132.59,5.35
YM2-SYNC  (via drill 0.35)
  Top 0.203: v122.68,4.57 123.19,4.57 124.46,5.84 SL1.10
  Bottom 0.152: 99.06,17.27 99.06,33.02 101.35,35.31 IC5.LOAD
  Bottom 0.203: IC4.SH 109.98,64.01 112.78,61.21 112.78,45.47 105.16,37.85 105.16,35.56 104.9,35.31 IC5.LOAD | 99.06,17.27 99.06,16.76 101.85,13.97 115.06,13.97 115.57,13.46 115.57,6.6 117.6,4.57 v122.68,4.57
YM3-CLK-O
  Bottom 0.203: IC7.SY 135.38,71.63 136.65,70.36 136.65,45.47 135.43,44.25 135.43,34.16 134.03,32.77 IC8.CLK 138.43,32.77 140.21,30.99 140.21,22.61 142.24,20.57 142.24,19.81 | 142.24,19.81 SL1.3 | 142.24,19.81
YM3-CS  (via drill 0.35)
  Top 0.203: U1.52 53.05,72.35 54.56,73.86 60.23,73.86 v60.83,73.27
  Bottom 0.203: v60.83,73.27 62.72,71.37 63.75,71.37 69.6,77.22 69.6,79.5 70.61,80.52 110.49,80.52 114.3,76.71 114.3,59.69 115.06,58.93 IC7./CS
YM3-OUTPUT
  Bottom 0.203: IC7.MO 134.87,66.55 136.14,65.28 136.14,45.47 128.63,37.95 128.63,35.41 IC8.SD 125.73,32.77 122.94,29.97 122.94,11.94 123.95,10.92 130.56,10.92 132.08,9.4 SL1.7
YM3-SYNC
  Bottom 0.152: 121.92,28.96 121.92,31.24 IC8.LOAD
  Bottom 0.203: IC7.SH 133.1,64.01 135.64,61.47 135.64,45.47 128.27,38.1 128.27,35.81 127.76,35.31 IC8.LOAD | SL1.11 121.92,28.96
YM4-CLK-O  (via drill 0.35)
  Top 0.203: v166.12,5.59 165.48,4.95 141.1,4.95 139.7,6.35 SL1.4
  Bottom 0.203: IC10.SY 156.72,71.63 157.99,70.36 157.99,43.43 158.5,42.93 158.5,33.53 157.73,32.77 IC11.CLK 160.27,32.77 168.66,24.38 168.66,15.24 | 168.66,15.24 168.66,8.13 v166.12,5.59 | 168.66,15.24
YM4-CS  (via drill 0.35)
  Top 0.203: U1.53 52.55,72.36 54.41,74.22 61.16,74.22 v61.47,73.91
  Bottom 0.203: v61.47,73.91 62.99,72.39 64.01,72.39 68.99,77.37 68.99,79.65 70.36,81.03 132.84,81.03 137.16,76.71 137.16,59.69 137.92,58.93 IC10./CS
YM4-OUTPUT  (via drill 0.35)
  Top 0.203: IC11.SD 144.73,28.65 144.73,24.09 139.82,19.18 v139.82,18.54
  Bottom 0.203: IC10.MO 156.72,66.55 157.48,65.79 157.48,43.94 151.49,37.95 151.49,35.15 149.1,32.77 IC11.SD | v139.82,18.54 139.82,16.89 134.62,11.68 133.6,11.68 133.35,11.43 133.35,7.62 132.08,6.35 130.3,6.35 129.54,7.11 SL1.8
YM4-SYNC  (via drill 0.35)
  Top 0.203: v138.68,18.54 138.93,18.79 138.93,18.8 144.37,24.24 144.37,30.84 IC11.LOAD | SL1.12 119.38,7.37 119.89,6.86 122.43,6.86 123.19,7.62 123.19,11.18 v124.46,12.45
  Bottom 0.203: IC10.SH 156.97,61.72 156.97,43.9 151.16,38.08 151.16,35.59 150.88,35.31 IC11.LOAD | v138.68,18.54 138.68,16.26 135.89,13.46 125.48,13.46 v124.46,12.45
YM-A0
  Top 0.203: U1.3 41.19,66.5 39.12,68.58 39.12,74.42 42.52,77.83 63.39,77.83 68.83,72.38 68.83,67.56 69.85,66.55 IC1.A0 83.64,66.55 84.81,67.72 88.42,67.72 89.58,66.55 IC4.A0 106.5,66.55 107.67,67.72 111.78,67.72 112.95,66.55 IC7.A0 129.11,66.55 130.28,67.72 134.39,67.72 135.56,66.55 IC10.A0
YM-CLK-I
  Top 0.203: IC10.M 142.16,74.17 140.74,72.75 136.63,72.75 135.21,74.17 IC7.M 119.3,74.17 117.88,72.75 114.28,72.75 112.85,74.17 IC4.M 96.19,74.17 95.02,73 91.67,73 90.5,74.17 IC1.M
  Bottom 0.203: IC14.6 168.4,66.8 168.4,74.17 166.37,76.2 159,76.2 156.97,74.17 IC10.M
YM-D0  (via drill 0.35)
  Top 0.203: U1.54 52.05,72.36 54.26,74.57 61.83,74.57 64.67,71.73 64.67,55.73 v64.65,55.73 | IC10.D0 137.41,51.31 133.6,47.5 123.44,47.5 119.63,51.31 IC7.D0 114.05,51.31 110.24,47.5 100.84,47.5 97.03,51.31 IC4.D0 91.36,51.31 87.4,47.35 77.63,47.35 73.67,51.31 IC1.D0
  Bottom 0.203: v64.65,55.73 64.65,54.73 65.02,54.36 66.29,54.36 67.25,53.4 | IC1.D0 69.34,51.31 67.25,53.4 | 67.25,53.4
YM-D1
  Top 0.203: U1.55 51.55,72.38 54.1,74.93 61.98,74.93 65.28,71.63 65.28,52.07 68.58,48.77 IC1.D1 72.9,48.77 77.22,44.45 87.63,44.45 91.95,48.77 IC4.D1 96.01,48.77 100.33,44.45 110.24,44.45 114.55,48.77 IC7.D1 118.36,48.77 122.68,44.45 132.84,44.45 137.16,48.77 IC10.D1
YM-D2
  Top 0.203: U1.56 51.05,72.38 53.95,75.29 62.21,75.29 65.79,71.71 65.79,53.34 69.09,50.04 73.15,50.04 76.96,46.23 IC1.D2 87.38,46.23 91.19,50.04 96.52,50.04 100.33,46.23 IC4.D2 110.49,46.23 114.3,50.04 119.13,50.04 122.94,46.23 IC7.D2 133.35,46.23 137.16,50.04 144.78,50.04 148.59,46.23 IC10.D2
YM-D3
  Top 0.203: U1.57 50.55,72.38 53.86,75.69 62.31,75.69 66.29,71.71 66.29,55.63 69.34,52.58 77.47,52.58 81.28,48.77 IC1.D3 89.92,52.58 99.82,52.58 103.63,48.77 IC4.D3 112.78,52.58 123.19,52.58 127,48.77 IC7.D3 135.38,52.32 145.03,52.32 148.59,48.77 IC10.D3
YM-D4
  Top 0.203: IC10.D4 149.1,51.31 145.29,55.12 135.64,55.12 IC7.D4 127.25,51.31 123.44,55.12 112.78,55.12 IC4.D4 104.14,51.31 100.33,55.12 89.92,55.12 IC1.D4 81.28,51.31 77.47,55.12 69.09,55.12 66.8,57.4 66.8,71.72 62.47,76.05 53.71,76.05 50.05,72.39 U1.58
YM-D5
  Top 0.203: U1.59 49.55,72.41 53.54,76.4 62.62,76.4 67.31,71.71 67.31,59.69 69.34,57.66 77.47,57.66 81.28,53.85 IC1.D5 89.92,57.66 100.84,57.66 104.65,53.85 IC4.D5 112.78,57.66 123.95,57.66 127.76,53.85 IC7.D5 135.64,57.66 146.05,57.66 149.86,53.85 IC10.D5
YM-D6
  Top 0.203: U1.61 48.51,69.49 48.51,71.88 53.39,76.76 62.77,76.76 67.67,71.86 67.67,62.48 69.85,60.3 79.39,60.3 83.31,56.39 IC1.D6 87.38,56.39 91.19,60.2 102.36,60.2 106.17,56.39 IC4.D6 110.24,56.39 113.79,59.94 125.73,59.94 129.29,56.39 IC7.D6 133.1,56.39 136.91,60.2 146.56,60.2 150.37,56.39 IC10.D6
YM-D7
  Top 0.203: U1.62 48.01,69.5 48.01,71.88 53.24,77.11 63.09,77.11 68.07,72.14 68.07,64.26 69.6,62.74 80.52,62.74 84.33,58.93 IC1.D7 90.07,62.89 102.46,62.89 106.43,58.93 IC4.D7 112.78,62.74 125.73,62.74 129.54,58.93 IC7.D7 135.64,62.74 147.07,62.74 150.88,58.93 IC10.D7
YM-RST
  Top 0.203: U1.4 41.15,66 38.73,68.42 38.73,74.55 42.37,78.18 63.53,78.18 69.19,72.53 69.19,69.85 69.95,69.09 IC1./IC 83.64,69.09 84.81,70.26 87.91,70.26 89.08,69.09 IC4./IC 106.5,69.09 107.93,70.51 110,70.51 111.43,69.09 IC7./IC 129.11,69.09 130.53,70.51 132.87,70.51 134.29,69.09 IC10./IC
YM-WR
  Top 0.203: U1.2 41.2,67 39.5,68.71 39.5,74.3 42.67,77.47 63.24,77.47 68.43,72.28 68.43,64.92 69.34,64.01 IC1./WR 83.31,64.01 84.73,65.43 88.75,65.43 90.17,64.01 IC4./WR 106.25,64.01 107.67,65.43 111.02,65.43 112.44,64.01 IC7./WR 129.36,64.01 130.79,65.43 133.12,65.43 134.54,64.01 IC10./WR

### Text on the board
tNames: SynthModule V1.0 - Brian Oehlers, Ruben van Renswoude en Julian Schotborgh

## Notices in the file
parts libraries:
SparkFun-Connectors: Licensing: Creative Commons ShareAlike 4.0 International - https://creativecommons.org/licenses/by-sa/4.0
LDO: License : GNU General Public License version 2 (see bottom)
